(* Logix 5000 AddOnInstructionDefinition export Banner_EZAK2_Param_v4; software revision 33.00 *)

TYPE Banner_EZAK2_Channel_States_v4 :   // Channel States for the EZ-Array.
STRUCT
   State_16_to_1 : INT;
   State_32_to_17 : INT;
   State_48_to_33 : INT;
   State_64_to_49 : INT;
   State_80_to_65 : INT;
   State_96_to_81 : INT;
   State_112_to_97 : INT;
   State_128_to_113 : INT;
   State_144_to_129 : INT;
   State_160_to_145 : INT;
   State_176_to_161 : INT;
   State_192_to_177 : INT;
   State_208_to_193 : INT;
   State_224_to_209 : INT;
   State_240_to_225 : INT;
   State_256_to_241 : INT;
   State_272_to_257 : INT;
   State_288_to_273 : INT;
   State_304_to_289 : INT;
   State_320_to_305 : INT;
   State_336_to_321 : INT;
   State_352_to_337 : INT;
   State_368_to_353 : INT;
   State_384_to_369 : INT;
   State_400_to_385 : INT;
   State_416_to_401 : INT;
   State_432_to_417 : INT;
   State_448_to_433 : INT;
   State_464_to_449 : INT;
   State_480_to_465 : INT;
END_STRUCT
END_TYPE

TYPE Banner_EZAK2_RD_v4 :   // UDT with all of the Read only parameters for EZ-Array.
STRUCT
   Master_Cycle_Time : INT;
   Min_Cycle_Time : INT;
   M_Sequence_Capability : INT;
   IO_Link_Version_ID : INT;
   Process_Data_Input_Length : INT;
   Process_Data_Output_Length : INT;
   Combined_Vendor_ID : DINT;   // IO-Link Vendor ID
   Vendor_ID1 : INT;
   Vendor_ID2 : INT;
   Combined_Device_ID : DINT;   // IO-Link Device ID
   Device_ID1 : INT;
   Device_ID2 : INT;
   Device_ID3 : INT;
   Measurement_1 : DINT;
   Measurement_2 : DINT;
   CS : Banner_EZAK2_Channel_States_v4;   // Channel States
   Number_of_Emitter_Channels : DINT;
   Emitter_First_Bad_Channel : DINT;
   Number_of_Receiver_Channels : DINT;
   Dip_Switch_6 : SINT;   // 0 = ON, 1 = OFF
   Dip_Switch_5 : SINT;   // 0 = ON, 1 = OFF
   Dip_Switch_4 : SINT;   // 0 = ON, 1 = OFF
   Dip_Switch_3 : SINT;   // 0 = ON, 1 = OFF
   Dip_Switch_2 : SINT;   // 0 = ON, 1 = OFF
   Dip_Switch_1 : SINT;   // 0 = ON, 1 = OFF
   Error_Code : SINT;   // See IODD file for Error Codes.
   Alignment_Status : SINT;   // 0 = Failed, 1 = Success
   Discrete_Output_1 : SINT;   // 0 = OFF, 1 = ON
   Discrete_Output_2 : SINT;   // 0 = OFF, 1 = ON
   Analog_Output_1_DAC_Value : DINT;
   Analog_Output_2_DAC_Value : DINT;
   First_Beam_Blocked : DINT;
   Last_Beam_Blocked : DINT;
   Total_Beam_Blocked : DINT;
   Transitions : DINT;
   Contiguous_Beam_Blocked : DINT;
   First_Beam_Made : DINT;
   Last_Beam_Made : DINT;
   Total_Beam_Made : DINT;
   Contiguous_Beam_Made : DINT;
   Middle_Beam_Blocked : DINT;
   Outer_Diameter : DINT;
   Inner_Diameter : DINT;
   Contiguous_First_Beam_Blocked : DINT;
   Contiguous_Last_Beam_Blocked : DINT;
   Object_1_First_Beam_Blocked : DINT;
   Object_1_Last_Beam_Blocked : DINT;
   Object_2_First_Beam_Blocked : DINT;
   Object_2_Last_Beam_Blocked : DINT;
   Object_3_First_Beam_Blocked : DINT;
   Object_3_Last_Beam_Blocked : DINT;
   Carpet_Nap : DINT;
   Analog_1_Latched : DINT;
   Analog_2_Latched : DINT;
   Carpet_Edge : DINT;
   Receiver_Firmware_Number : DINT;
   Receiver_Firmware_Version : SINT;
   Emitter_Firmware_Number : DINT;
   Emitter_Firmware_Version : SINT;
   Communications_Fimware_Number : DINT;
   Communications_Firmware_Version : SINT;
END_STRUCT
END_TYPE

TYPE Banner_EZAK2_v4 :   // UDT with all of the parameters for EZ-Array.
STRUCT
   Initial_Global_Read : BOOL;   // Determines if all of the IO-Link data has been read into the PLC yet
   Command : INT;   // Value placed in here will activate a read or write to a specifc IO-Link Index
   Read : Banner_EZAK2_RD_v4;   // All read data
   Write : Banner_EZAK2_WD_v4;   // All data that can be written to.
   Archive_Data : Banner_EZAK2_WD_v4;
   Reset : BOOL;   // Resets AOI. This will force a complete parameter read of the sensor.
END_STRUCT
END_TYPE

TYPE Banner_EZAK2_WD_v4 :   // UDT that stores the Write Data for a EZ-Array.
STRUCT
   System_Command : INT;   // 130 = Factory Reset.
   Parameter_Access_Lock : SINT;
   Data_Storage_Lock : SINT;
   Local_Parameterization_Lock : SINT;
   Local_User_Interface_Lock : SINT;
   Scan_Type : INT;   // 1 = Straight, 2 = Single Edge, 3 = Double Edge (DE), 4 = DE Step 2, 5 = DE Step 4, 6 = DE Step 8, 7 = DE Step 16, 8=DE Step 32, 10 = Carpet Nap.
   Remote_Teach : INT;
   Blanking : Banner_EZAK2_Channel_States_v4;   // Status of Beam Banking
   Reserved : INT;
   Gain_Method : SINT;   // 1 = High Excess, 2 = Low Contrast
   Low_Contrast_Sensitivity : INT;
   Display_Orientation : SINT;   // 0 = Normal Orientation, 1 = Inverted Orientation
   Configuration_Type : SINT;   // 0 = Dip Switch Control, 1 = Advanced Control
   Sensitivity_Button : SINT;   // 0 = Enabled, 1 = Disabled
   Align_Blank_Button : SINT;   // 0 = Enabled, 1 = Disabled
   Measurement_1 : INT;   // 0=Disabled, 1=FBB, 2=LBB, 3=TBB, 4=TRN, 5=CBB, 6=FBM, 7=LBM, 8=TBM, 9=CBM, 10=MBB, 11=OD, 12=ID, 13=CFBB, 14=CLBB, 15=O1 FBB, 16=O1 LBB, 17=O2 FBB, 18=O2 LBB, 19=O3 FBB, 20=O3 LBB, 21=Carpet Nap, 24=Carpet Edge.
   Measurement_2 : INT;   // 0=Disabled, 1=FBB, 2=LBB, 3=TBB, 4=TRN, 5=CBB, 6=FBM, 7=LBM, 8=TBM, 9=CBM, 10=MBB, 11=OD, 12=ID, 13=CFBB, 14=CLBB, 15=O1 FBB, 16=O1 LBB, 17=O2 FBB, 18=O2 LBB, 19=O3 FBB, 20=O3 LBB, 21=Carpet Nap, 24=Carpet Edge.
   Number_of_Dirty_Channels : DINT;
   Time_of_Service : DINT;
   Alignment_Blanking_Mode : INT;   // 0=Status:Idle Mode, 1=Enter Align State, 2=Status:Align Mode, 3=Exit Align State, 4=Enter Blanking State, 5=Status: Blanking Mode, 6=Exit Blanking Mode.
   DO1_Status : SINT;   // 0 = Disabled, 1 = Enabled
   DO1_Type : SINT;   // 0 = Measurement Mode, 1 = Alarm or Health Mode
   DO1_Mode : SINT;   // 0 = NC (Alarm), 1 = NO (Health)
   DO1_Measurement : SINT;   // 0 = Measurement 2, 1 = Measurement 1
   DO1_Scan_Response : INT;   // See IODD for range.
   DO1_Hysteresis_Low : INT;   // See IODD for range.
   DO1_Hysteresis_High : INT;   // See IODD for range.
   DO1_Threshold_Low : INT;   // See IODD for range.
   DO1_Threshold_High : INT;   // See IODD for range.
   DO2_Status : SINT;   // 0 = Disabled, 1 = Enabled
   DO2_Type : SINT;   // 0 = Measurement Mode, 1 = Alarm or Health Mode
   DO2_Mode : SINT;   // 0 = NC (Alarm), 1 = NO (Health)
   DO2_Measurement : SINT;   // 0 = Measurement 2, 1 = Measurement 1
   DO2_Scan_Response : INT;   // See IODD for range.
   DO2_Hysteresis_Low : INT;   // See IODD for range.
   DO2_Hysteresis_High : INT;   // See IODD for range.
   DO2_Threshold_Low : INT;   // See IODD for range.
   DO2_Threshold_HIgh : INT;   // See IODD for range.
   Emitter_Power : INT;   // 1 to 11
   User_Process_Data : INT;   // 0 = Active Measurements, 1= Straight Scan, 2 = Single Double Edge, 128 = Channel States OR, 129 = Channel States AND.
   IO_Com : SINT;   // Allows for change between COM2 and Com3 Operation.
END_STRUCT
END_TYPE

TYPE Banner_IOL_Port_v4 :   // UDT that has all of the data items necessary to communicate with a specific Port on a IO-Link Master
STRUCT
   Port_Controlled : INT;   // Each bit represents a port on an IO-Link Master. Set to 1 to tell AOI to control that port.
   Port_Activate : INT;   // Each bit represents a port on an IO-Link Master. When ON that port will process any commands in queue.
   Port_Read : INT;   // Each bit represents a port on an IO-Link Master. Used to determine when device AOI has requested a Read command.
   Port_Write : INT;   // Each bit represents a port on an IO-Link Master. Used to determine when device AOI has requested a Write command.
   Port_RW_Complete : INT;   // Each bit represents a port on an IO-Link Master. Tells device AOI that Read or Write request has been completed.
   Port_Device_Read : INT;
   Data_Transfer : SINT[190];   // Array to transfer data from IO-Master to device AOIs.
END_STRUCT
END_TYPE

ADD_ON_INSTRUCTION Banner_EZAK2_Param_v4   (* revision 4.1, vendor Banner Engineering *)
// AOI to read and write parameter data to an IO-Link EZ-Array K2.
// Revision note:
// Fixed Alignment Blanking mode byte order for write. Switched System command from SINT to INT.
VAR_IN_OUT
   EZAK2 : Banner_EZAK2_v4; {required}
   Port_Data : Banner_IOL_Port_v4; {required}
END_VAR
VAR_INPUT
   Port : DINT; {required}
END_VAR
VAR
   Local_Control : DINT; {access None}
   Global_Read_Command_Value : INT; {access None}
   Global_Write_Command_Value : INT; {access None}
   Command_Being_Processed : BOOL; {access None}
   Update_Archive : BOOL; {access None}
   Index_Write_Control : DINT; {access None}
   Index_Write_Inprocess : INT; {access None}
   Inprocess_Index : DINT; {access None}
END_VAR

ROUTINE Logic   (* ladder *)
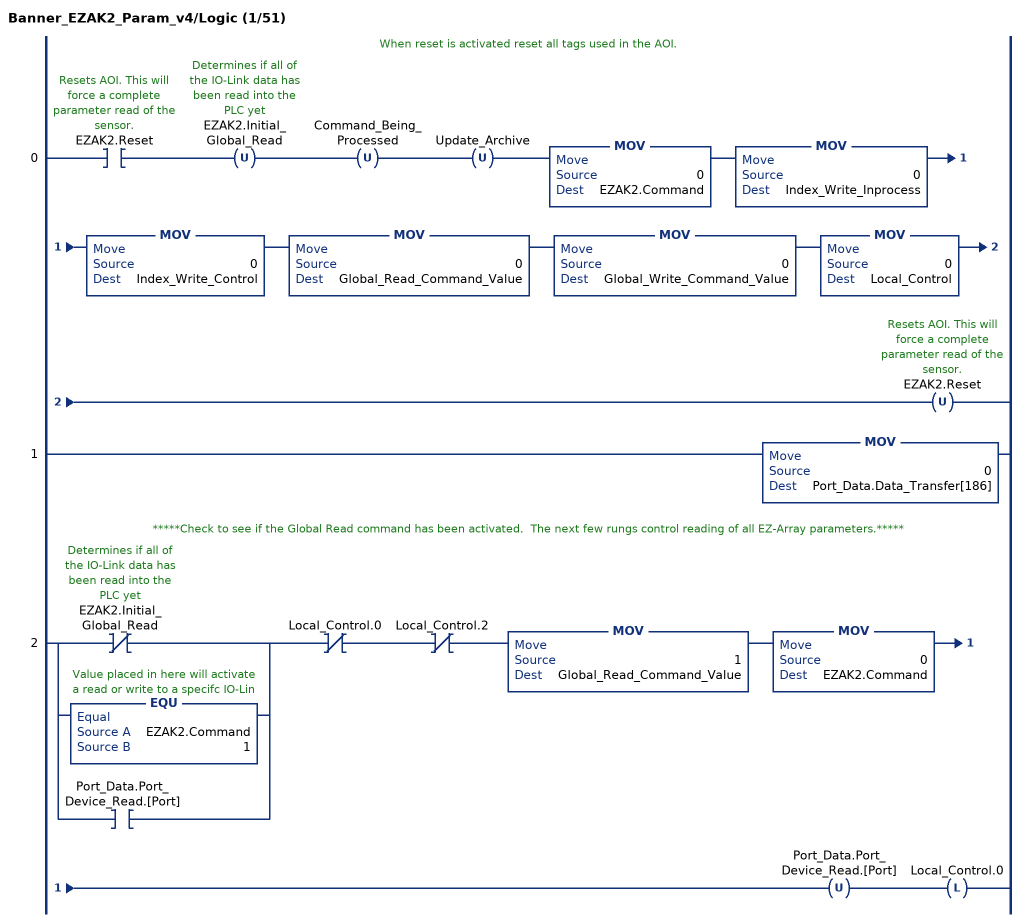
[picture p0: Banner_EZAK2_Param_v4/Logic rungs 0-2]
   // When reset is activated reset all tags used in the AOI.
   0: XIC(EZAK2.Reset)OTU(EZAK2.Initial_Global_Read)OTU(Command_Being_Processed)OTU(Update_Archive)MOV(0,EZAK2.Command)MOV(0,Index_Write_Inprocess)MOV(0,Index_Write_Control)MOV(0,Global_Read_Command_Value)MOV(0,Global_Write_Command_Value)MOV(0,Local_Control)OTU(EZAK2.Reset);
   1: MOV(0,Port_Data.Data_Transfer[186]);
   // *****Check to see if the Global Read command has been activated.  The next few rungs control reading of all EZ-Array parameters.*****
   2: [XIO(EZAK2.Initial_Global_Read) ,EQU(EZAK2.Command,1) ,XIC(Port_Data.Port_Device_Read.[Port]) ]XIO(Local_Control.0)XIO(Local_Control.2)MOV(1,Global_Read_Command_Value)MOV(0,EZAK2.Command)OTU(Port_Data.Port_Device_Read.[Port])OTL(Local_Control.0);
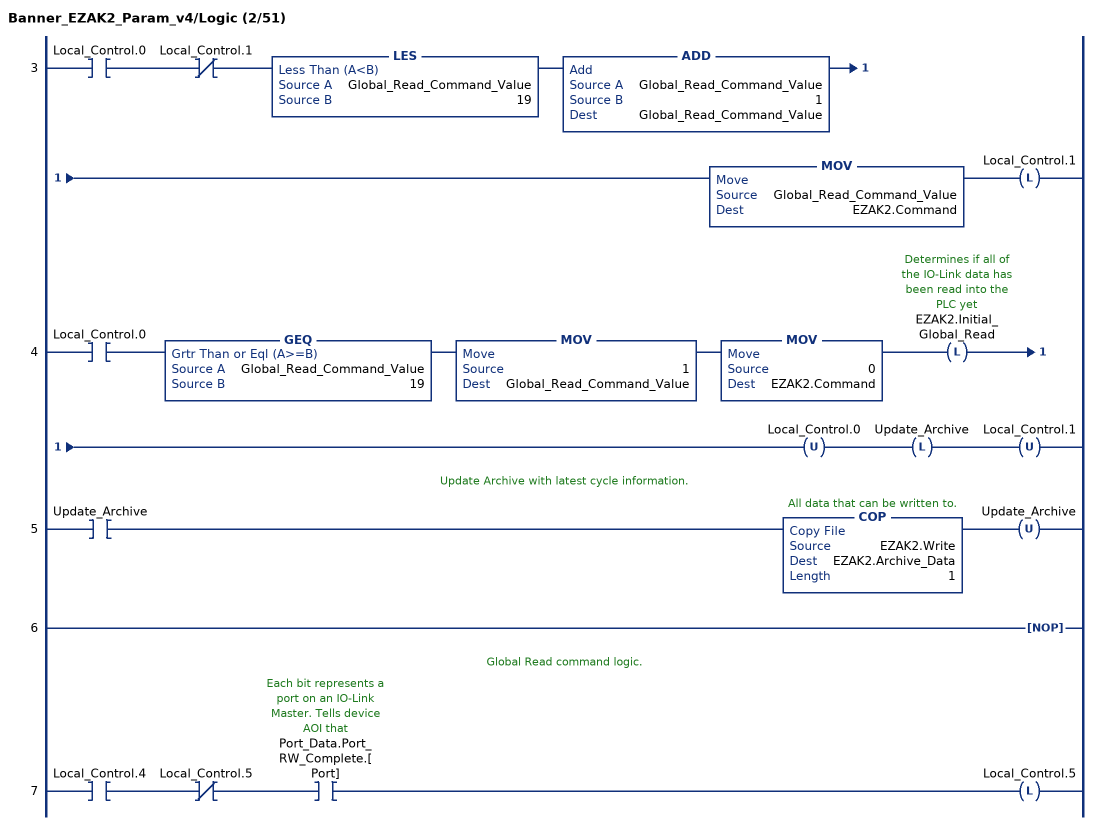
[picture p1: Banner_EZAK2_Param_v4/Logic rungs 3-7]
   3: XIC(Local_Control.0)XIO(Local_Control.1)LES(Global_Read_Command_Value,19)ADD(Global_Read_Command_Value,1,Global_Read_Command_Value)MOV(Global_Read_Command_Value,EZAK2.Command)OTL(Local_Control.1);
   4: XIC(Local_Control.0)GEQ(Global_Read_Command_Value,19)MOV(1,Global_Read_Command_Value)MOV(0,EZAK2.Command)OTL(EZAK2.Initial_Global_Read)OTU(Local_Control.0)OTL(Update_Archive)OTU(Local_Control.1);
   // Update Archive with latest cycle information.
   5: XIC(Update_Archive)COP(EZAK2.Write,EZAK2.Archive_Data,1)OTU(Update_Archive);
   6: NOP();
   // Global Read command logic.
   7: XIC(Local_Control.4)XIO(Local_Control.5)XIC(Port_Data.Port_RW_Complete.[Port])OTL(Local_Control.5);
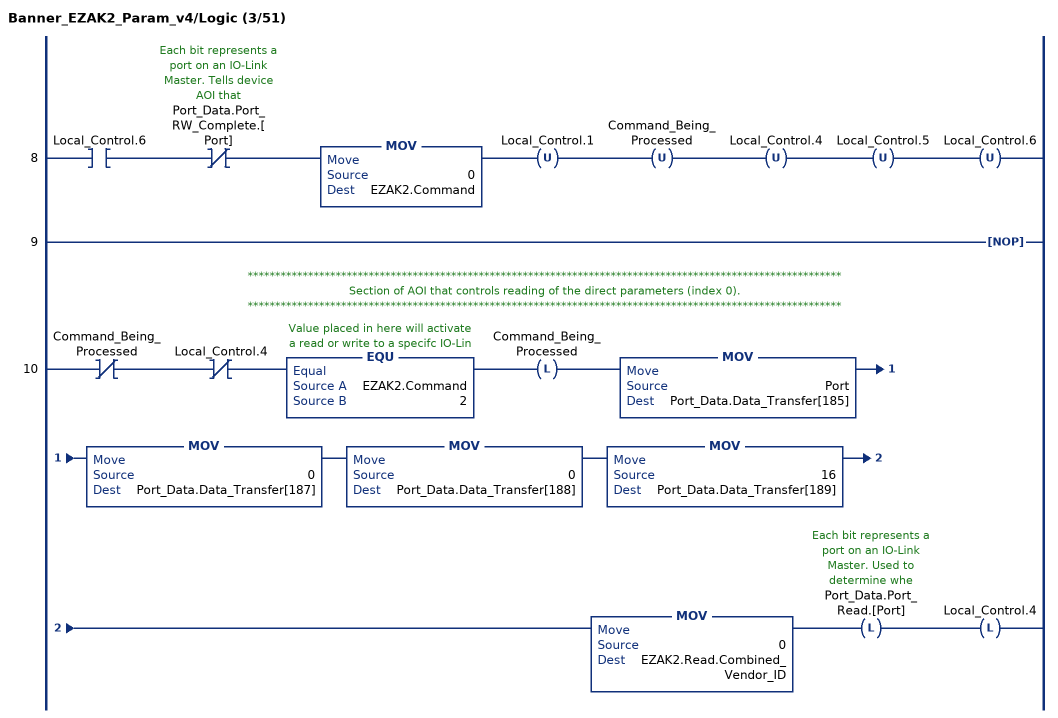
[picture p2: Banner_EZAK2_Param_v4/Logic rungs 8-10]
   8: XIC(Local_Control.6)XIO(Port_Data.Port_RW_Complete.[Port])MOV(0,EZAK2.Command)OTU(Local_Control.1)OTU(Command_Being_Processed)OTU(Local_Control.4)OTU(Local_Control.5)OTU(Local_Control.6);
   9: NOP();
   // ************************************************************************************************************
   // Section of AOI that controls reading of the direct parameters (index 0).
   // ************************************************************************************************************
   10: XIO(Command_Being_Processed)XIO(Local_Control.4)EQU(EZAK2.Command,2)OTL(Command_Being_Processed)MOV(Port,Port_Data.Data_Transfer[185])MOV(0,Port_Data.Data_Transfer[187])MOV(0,Port_Data.Data_Transfer[188])MOV(16,Port_Data.Data_Transfer[189])MOV(0,EZAK2.Read.Combined_Vendor_ID)OTL(Port_Data.Port_Read.[Port])OTL(Local_Control.4);
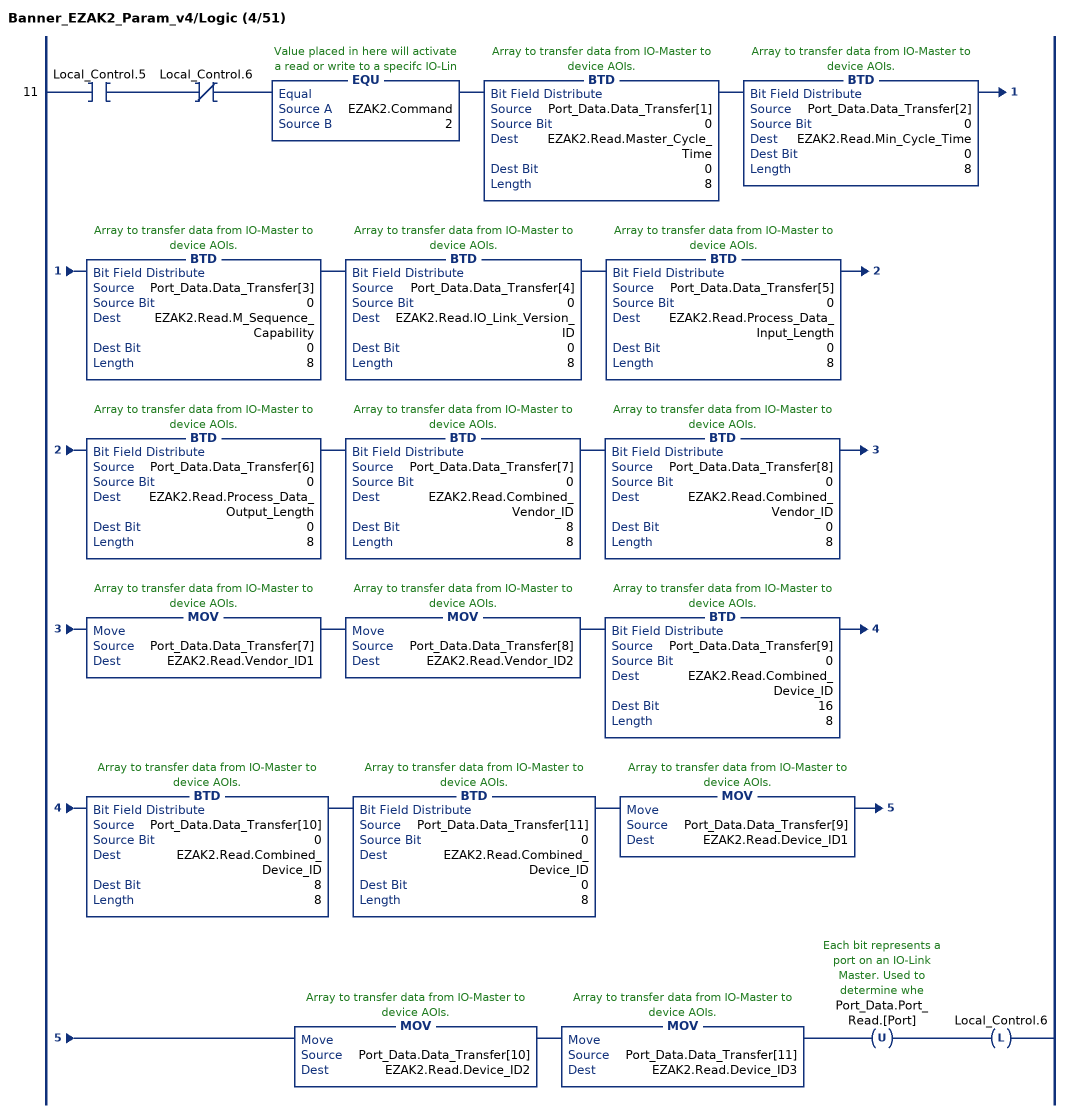
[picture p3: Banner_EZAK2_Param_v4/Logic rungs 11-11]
   11: XIC(Local_Control.5)XIO(Local_Control.6)EQU(EZAK2.Command,2)BTD(Port_Data.Data_Transfer[1],0,EZAK2.Read.Master_Cycle_Time,0,8)BTD(Port_Data.Data_Transfer[2],0,EZAK2.Read.Min_Cycle_Time,0,8)BTD(Port_Data.Data_Transfer[3],0,EZAK2.Read.M_Sequence_Capability,0,8)BTD(Port_Data.Data_Transfer[4],0,EZAK2.Read.IO_Link_Version_ID,0,8)BTD(Port_Data.Data_Transfer[5],0,EZAK2.Read.Process_Data_Input_Length,0,8)BTD(Port_Data.Data_Transfer[6],0,EZAK2.Read.Process_Data_Output_Length,0,8)BTD(Port_Data.Data_Transfer[7],0,EZAK2.Read.Combined_Vendor_ID,8,8)BTD(Port_Data.Data_Transfer[8],0,EZAK2.Read.Combined_Vendor_ID,0,8)MOV(Port_Data.Data_Transfer[7],EZAK2.Read.Vendor_ID1)MOV(Port_Data.Data_Transfer[8],EZAK2.Read.Vendor_ID2)BTD(Port_Data.Data_Transfer[9],0,EZAK2.Read.Combined_Device_ID,16,8)BTD(Port_Data.Data_Transfer[10],0,EZAK2.Read.Combined_Device_ID,8,8)BTD(Port_Data.Data_Transfer[11],0,EZAK2.Read.Combined_Device_ID,0,8)MOV(Port_Data.Data_Transfer[9],EZAK2.Read.Device_ID1)MOV(Port_Data.Data_Transfer[10],EZAK2.Read.Device_ID2)MOV(Port_Data.Data_Transfer[11],EZAK2.Read.Device_ID3)OTU(Port_Data.Port_Read.[Port])OTL(Local_Control.6);
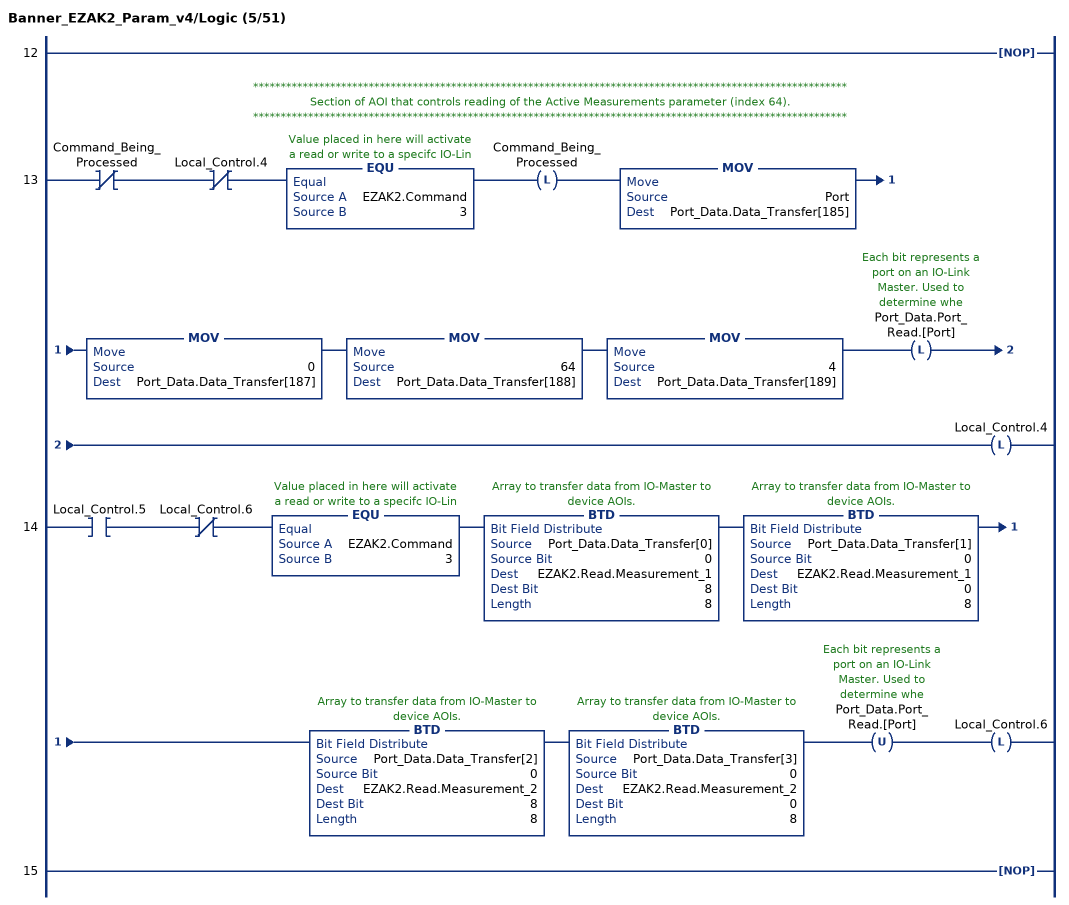
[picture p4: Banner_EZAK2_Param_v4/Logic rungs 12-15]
   12: NOP();
   // ************************************************************************************************************
   // Section of AOI that controls reading of the Active Measurements parameter (index 64).
   // ************************************************************************************************************
   13: XIO(Command_Being_Processed)XIO(Local_Control.4)EQU(EZAK2.Command,3)OTL(Command_Being_Processed)MOV(Port,Port_Data.Data_Transfer[185])MOV(0,Port_Data.Data_Transfer[187])MOV(64,Port_Data.Data_Transfer[188])MOV(4,Port_Data.Data_Transfer[189])OTL(Port_Data.Port_Read.[Port])OTL(Local_Control.4);
   14: XIC(Local_Control.5)XIO(Local_Control.6)EQU(EZAK2.Command,3)BTD(Port_Data.Data_Transfer[0],0,EZAK2.Read.Measurement_1,8,8)BTD(Port_Data.Data_Transfer[1],0,EZAK2.Read.Measurement_1,0,8)BTD(Port_Data.Data_Transfer[2],0,EZAK2.Read.Measurement_2,8,8)BTD(Port_Data.Data_Transfer[3],0,EZAK2.Read.Measurement_2,0,8)OTU(Port_Data.Port_Read.[Port])OTL(Local_Control.6);
   15: NOP();
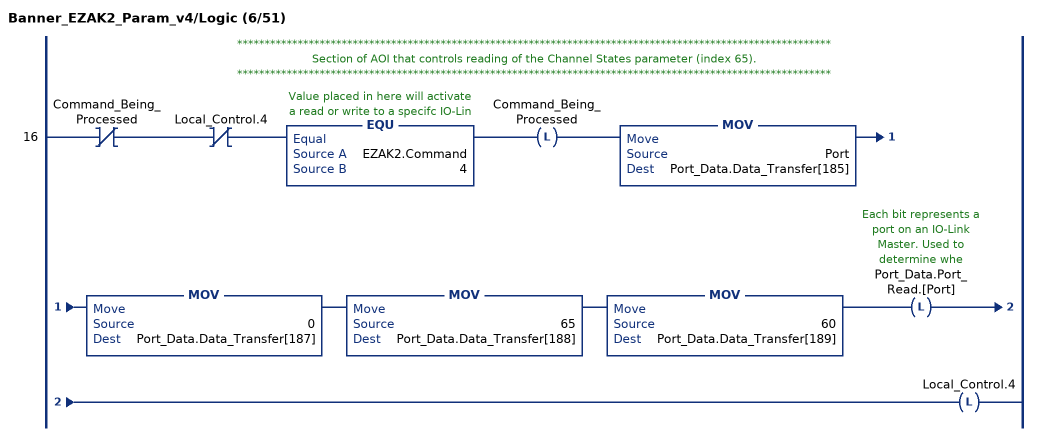
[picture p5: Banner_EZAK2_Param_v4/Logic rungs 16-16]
   // ************************************************************************************************************
   // Section of AOI that controls reading of the Channel States parameter (index 65).
   // ************************************************************************************************************
   16: XIO(Command_Being_Processed)XIO(Local_Control.4)EQU(EZAK2.Command,4)OTL(Command_Being_Processed)MOV(Port,Port_Data.Data_Transfer[185])MOV(0,Port_Data.Data_Transfer[187])MOV(65,Port_Data.Data_Transfer[188])MOV(60,Port_Data.Data_Transfer[189])OTL(Port_Data.Port_Read.[Port])OTL(Local_Control.4);
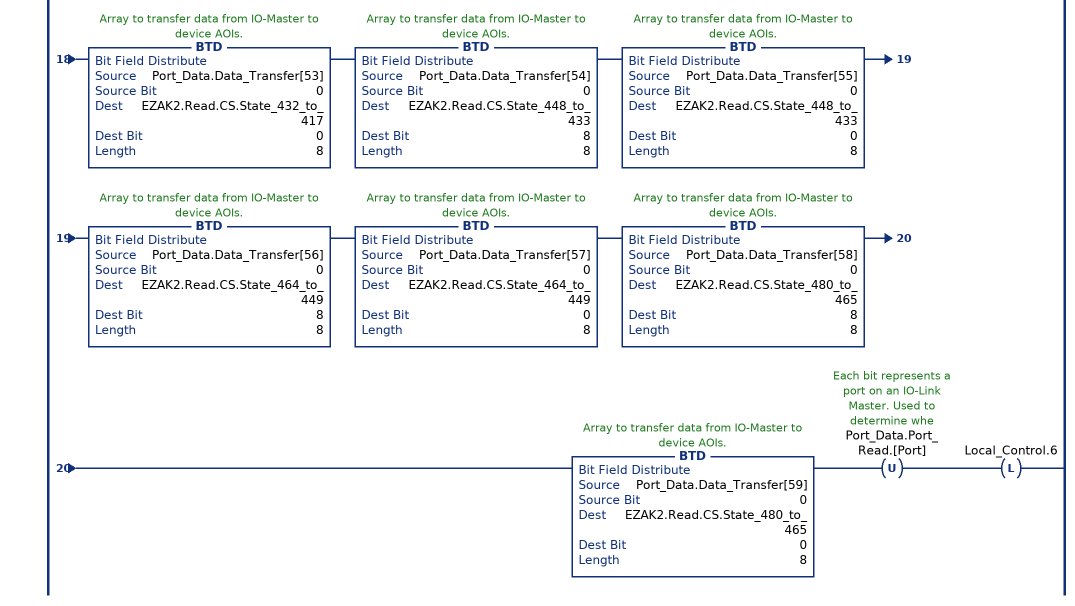
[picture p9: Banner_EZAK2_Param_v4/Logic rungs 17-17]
   17: XIC(Local_Control.5)XIO(Local_Control.6)EQU(EZAK2.Command,4)BTD(Port_Data.Data_Transfer[0],0,EZAK2.Read.CS.State_16_to_1,8,8)BTD(Port_Data.Data_Transfer[1],0,EZAK2.Read.CS.State_16_to_1,0,8)BTD(Port_Data.Data_Transfer[2],0,EZAK2.Read.CS.State_32_to_17,8,8)BTD(Port_Data.Data_Transfer[3],0,EZAK2.Read.CS.State_32_to_17,0,8)BTD(Port_Data.Data_Transfer[4],0,EZAK2.Read.CS.State_48_to_33,8,8)BTD(Port_Data.Data_Transfer[5],0,EZAK2.Read.CS.State_48_to_33,0,8)BTD(Port_Data.Data_Transfer[6],0,EZAK2.Read.CS.State_64_to_49,8,8)BTD(Port_Data.Data_Transfer[7],0,EZAK2.Read.CS.State_64_to_49,0,8)BTD(Port_Data.Data_Transfer[8],0,EZAK2.Read.CS.State_80_to_65,8,8)BTD(Port_Data.Data_Transfer[9],0,EZAK2.Read.CS.State_80_to_65,0,8)BTD(Port_Data.Data_Transfer[10],0,EZAK2.Read.CS.State_96_to_81,8,8)BTD(Port_Data.Data_Transfer[11],0,EZAK2.Read.CS.State_96_to_81,0,8)BTD(Port_Data.Data_Transfer[12],0,EZAK2.Read.CS.State_112_to_97,8,8)BTD(Port_Data.Data_Transfer[13],0,EZAK2.Read.CS.State_112_to_97,0,8)BTD(Port_Data.Data_Transfer[14],0,EZAK2.Read.CS.State_128_to_113,8,8)BTD(Port_Data.Data_Transfer[15],0,EZAK2.Read.CS.State_128_to_113,0,8)BTD(Port_Data.Data_Transfer[16],0,EZAK2.Read.CS.State_144_to_129,8,8)BTD(Port_Data.Data_Transfer[17],0,EZAK2.Read.CS.State_144_to_129,0,8)BTD(Port_Data.Data_Transfer[18],0,EZAK2.Read.CS.State_160_to_145,8,8)BTD(Port_Data.Data_Transfer[19],0,EZAK2.Read.CS.State_160_to_145,0,8)BTD(Port_Data.Data_Transfer[20],0,EZAK2.Read.CS.State_176_to_161,8,8)BTD(Port_Data.Data_Transfer[21],0,EZAK2.Read.CS.State_176_to_161,0,8)BTD(Port_Data.Data_Transfer[22],0,EZAK2.Read.CS.State_192_to_177,8,8)BTD(Port_Data.Data_Transfer[23],0,EZAK2.Read.CS.State_192_to_177,0,8)BTD(Port_Data.Data_Transfer[24],0,EZAK2.Read.CS.State_208_to_193,8,8)BTD(Port_Data.Data_Transfer[25],0,EZAK2.Read.CS.State_208_to_193,0,8)BTD(Port_Data.Data_Transfer[26],0,EZAK2.Read.CS.State_224_to_209,8,8)BTD(Port_Data.Data_Transfer[27],0,EZAK2.Read.CS.State_224_to_209,0,8)BTD(Port_Data.Data_Transfer[28],0,EZAK2.Read.CS.State_240_to_225,8,8)BTD(Port_Data.Data_Transfer[29],0,EZAK2.Read.CS.State_240_to_225,0,8)BTD(Port_Data.Data_Transfer[30],0,EZAK2.Read.CS.State_256_to_241,8,8)BTD(Port_Data.Data_Transfer[31],0,EZAK2.Read.CS.State_256_to_241,0,8)BTD(Port_Data.Data_Transfer[32],0,EZAK2.Read.CS.State_272_to_257,8,8)BTD(Port_Data.Data_Transfer[33],0,EZAK2.Read.CS.State_272_to_257,0,8)BTD(Port_Data.Data_Transfer[34],0,EZAK2.Read.CS.State_288_to_273,8,8)BTD(Port_Data.Data_Transfer[35],0,EZAK2.Read.CS.State_288_to_273,0,8)BTD(Port_Data.Data_Transfer[36],0,EZAK2.Read.CS.State_304_to_289,8,8)BTD(Port_Data.Data_Transfer[37],0,EZAK2.Read.CS.State_304_to_289,0,8)BTD(Port_Data.Data_Transfer[38],0,EZAK2.Read.CS.State_320_to_305,8,8)BTD(Port_Data.Data_Transfer[39],0,EZAK2.Read.CS.State_320_to_305,0,8)BTD(Port_Data.Data_Transfer[40],0,EZAK2.Read.CS.State_336_to_321,8,8)BTD(Port_Data.Data_Transfer[41],0,EZAK2.Read.CS.State_336_to_321,0,8)BTD(Port_Data.Data_Transfer[42],0,EZAK2.Read.CS.State_352_to_337,8,8)BTD(Port_Data.Data_Transfer[43],0,EZAK2.Read.CS.State_352_to_337,0,8)BTD(Port_Data.Data_Transfer[44],0,EZAK2.Read.CS.State_368_to_353,8,8)BTD(Port_Data.Data_Transfer[45],0,EZAK2.Read.CS.State_368_to_353,0,8)BTD(Port_Data.Data_Transfer[46],0,EZAK2.Read.CS.State_384_to_369,8,8)BTD(Port_Data.Data_Transfer[47],0,EZAK2.Read.CS.State_384_to_369,0,8)BTD(Port_Data.Data_Transfer[48],0,EZAK2.Read.CS.State_400_to_385,8,8)BTD(Port_Data.Data_Transfer[49],0,EZAK2.Read.CS.State_400_to_385,0,8)BTD(Port_Data.Data_Transfer[50],0,EZAK2.Read.CS.State_416_to_401,8,8)BTD(Port_Data.Data_Transfer[51],0,EZAK2.Read.CS.State_416_to_401,0,8)BTD(Port_Data.Data_Transfer[52],0,EZAK2.Read.CS.State_432_to_417,8,8)BTD(Port_Data.Data_Transfer[53],0,EZAK2.Read.CS.State_432_to_417,0,8)BTD(Port_Data.Data_Transfer[54],0,EZAK2.Read.CS.State_448_to_433,8,8)BTD(Port_Data.Data_Transfer[55],0,EZAK2.Read.CS.State_448_to_433,0,8)BTD(Port_Data.Data_Transfer[56],0,EZAK2.Read.CS.State_464_to_449,8,8)BTD(Port_Data.Data_Transfer[57],0,EZAK2.Read.CS.State_464_to_449,0,8)BTD(Port_Data.Data_Transfer[58],0,EZAK2.Read.CS.State_480_to_465,8,8)BTD(Port_Data.Data_Transfer[59],0,EZAK2.Read.CS.State_480_to_465,0,8)OTU(Port_Data.Port_Read.[Port])OTL(Local_Control.6);
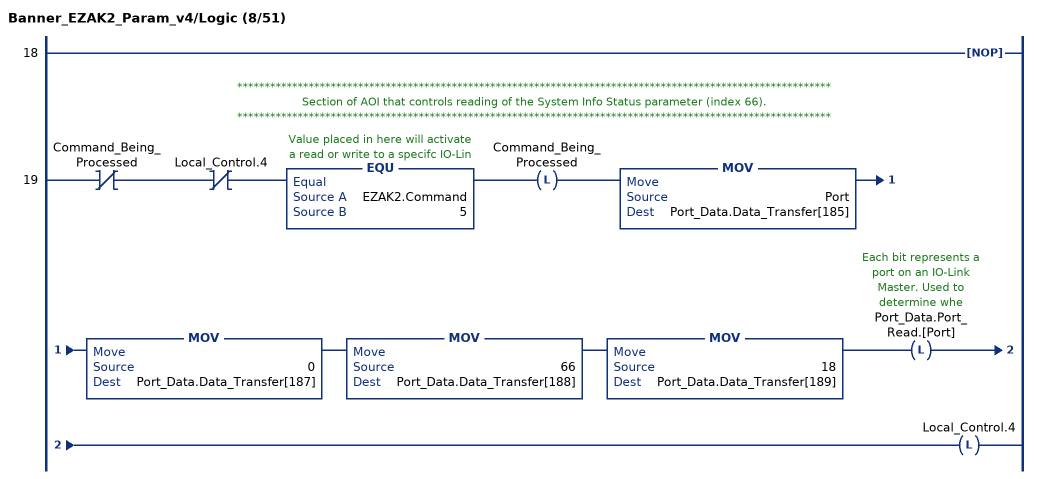
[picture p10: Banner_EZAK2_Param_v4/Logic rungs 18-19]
   18: NOP();
   // ************************************************************************************************************
   // Section of AOI that controls reading of the System Info Status parameter (index 66).
   // ************************************************************************************************************
   19: XIO(Command_Being_Processed)XIO(Local_Control.4)EQU(EZAK2.Command,5)OTL(Command_Being_Processed)MOV(Port,Port_Data.Data_Transfer[185])MOV(0,Port_Data.Data_Transfer[187])MOV(66,Port_Data.Data_Transfer[188])MOV(18,Port_Data.Data_Transfer[189])OTL(Port_Data.Port_Read.[Port])OTL(Local_Control.4);
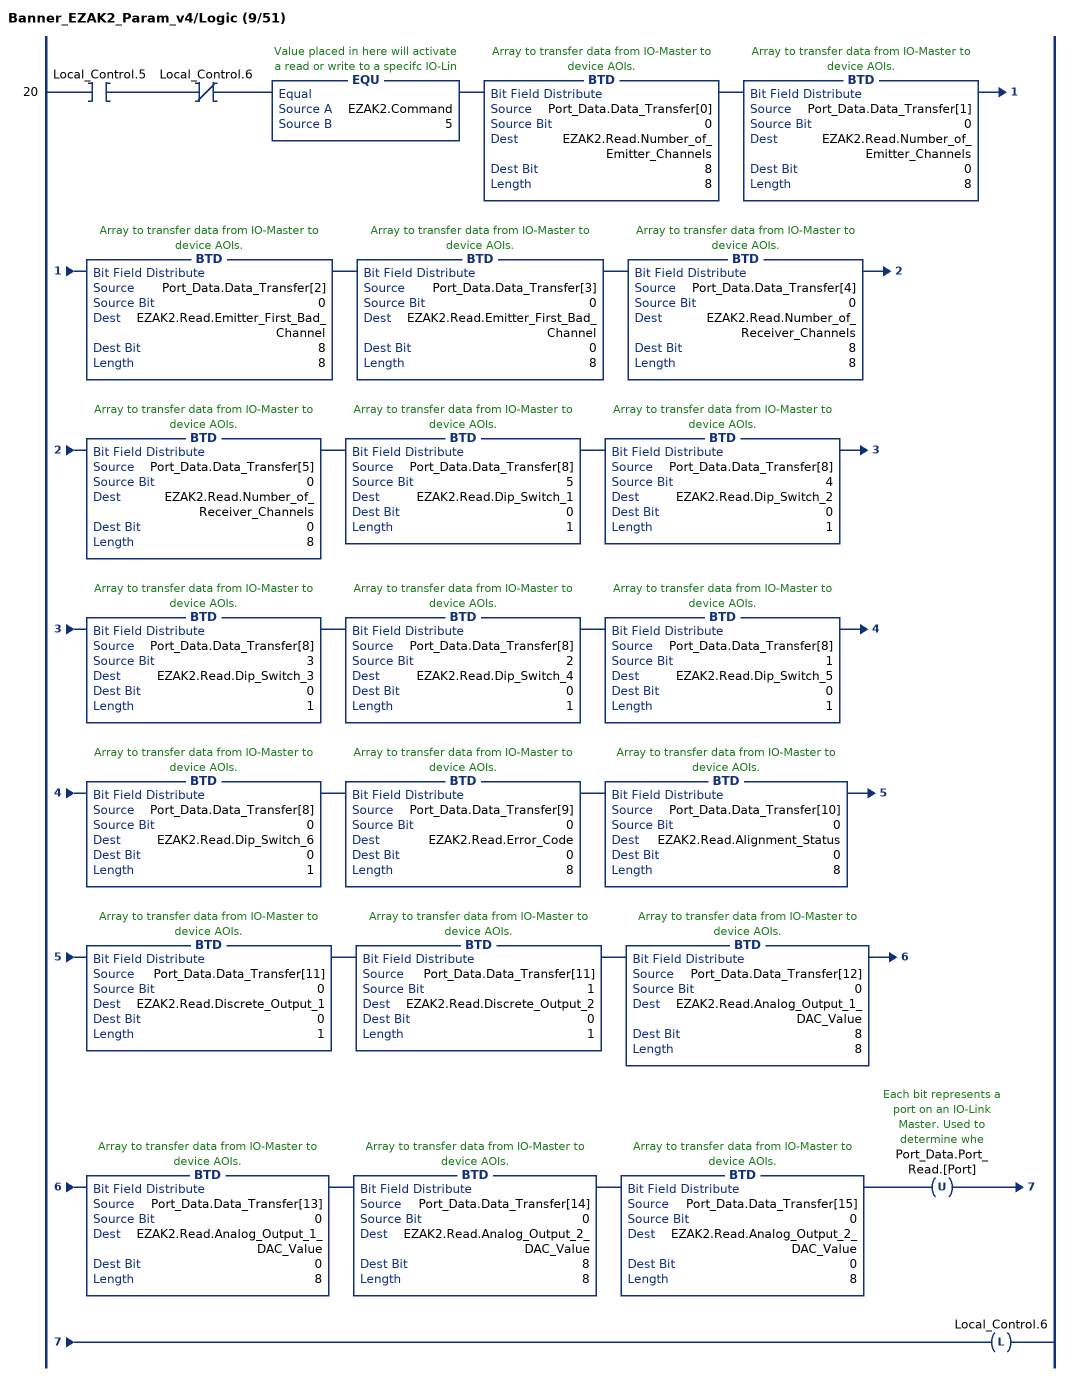
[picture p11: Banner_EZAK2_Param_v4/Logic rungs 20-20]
   20: XIC(Local_Control.5)XIO(Local_Control.6)EQU(EZAK2.Command,5)BTD(Port_Data.Data_Transfer[0],0,EZAK2.Read.Number_of_Emitter_Channels,8,8)BTD(Port_Data.Data_Transfer[1],0,EZAK2.Read.Number_of_Emitter_Channels,0,8)BTD(Port_Data.Data_Transfer[2],0,EZAK2.Read.Emitter_First_Bad_Channel,8,8)BTD(Port_Data.Data_Transfer[3],0,EZAK2.Read.Emitter_First_Bad_Channel,0,8)BTD(Port_Data.Data_Transfer[4],0,EZAK2.Read.Number_of_Receiver_Channels,8,8)BTD(Port_Data.Data_Transfer[5],0,EZAK2.Read.Number_of_Receiver_Channels,0,8)BTD(Port_Data.Data_Transfer[8],5,EZAK2.Read.Dip_Switch_1,0,1)BTD(Port_Data.Data_Transfer[8],4,EZAK2.Read.Dip_Switch_2,0,1)BTD(Port_Data.Data_Transfer[8],3,EZAK2.Read.Dip_Switch_3,0,1)BTD(Port_Data.Data_Transfer[8],2,EZAK2.Read.Dip_Switch_4,0,1)BTD(Port_Data.Data_Transfer[8],1,EZAK2.Read.Dip_Switch_5,0,1)BTD(Port_Data.Data_Transfer[8],0,EZAK2.Read.Dip_Switch_6,0,1)BTD(Port_Data.Data_Transfer[9],0,EZAK2.Read.Error_Code,0,8)BTD(Port_Data.Data_Transfer[10],0,EZAK2.Read.Alignment_Status,0,8)BTD(Port_Data.Data_Transfer[11],0,EZAK2.Read.Discrete_Output_1,0,1)BTD(Port_Data.Data_Transfer[11],1,EZAK2.Read.Discrete_Output_2,0,1)BTD(Port_Data.Data_Transfer[12],0,EZAK2.Read.Analog_Output_1_DAC_Value,8,8)BTD(Port_Data.Data_Transfer[13],0,EZAK2.Read.Analog_Output_1_DAC_Value,0,8)BTD(Port_Data.Data_Transfer[14],0,EZAK2.Read.Analog_Output_2_DAC_Value,8,8)BTD(Port_Data.Data_Transfer[15],0,EZAK2.Read.Analog_Output_2_DAC_Value,0,8)OTU(Port_Data.Port_Read.[Port])OTL(Local_Control.6);
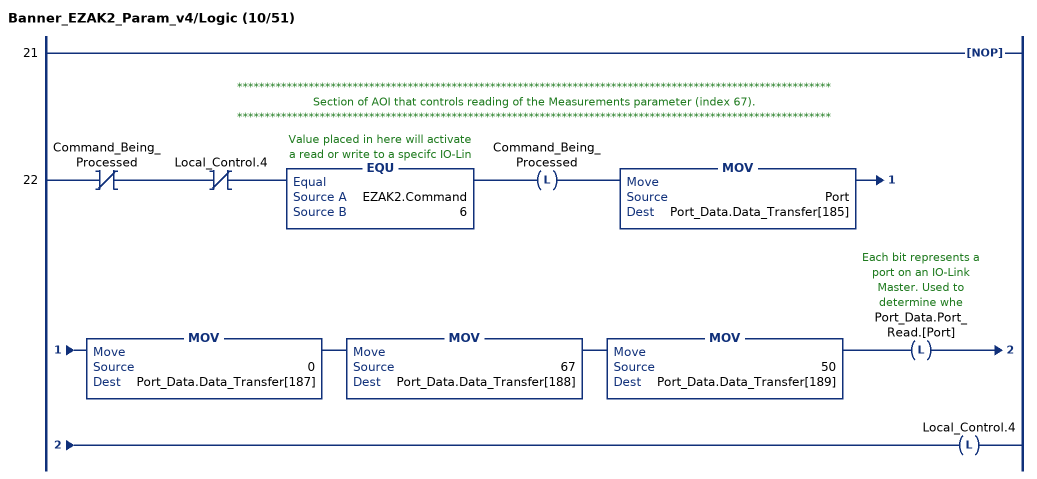
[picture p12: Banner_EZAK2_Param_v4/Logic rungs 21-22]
   21: NOP();
   // ************************************************************************************************************
   // Section of AOI that controls reading of the Measurements parameter (index 67).
   // ************************************************************************************************************
   22: XIO(Command_Being_Processed)XIO(Local_Control.4)EQU(EZAK2.Command,6)OTL(Command_Being_Processed)MOV(Port,Port_Data.Data_Transfer[185])MOV(0,Port_Data.Data_Transfer[187])MOV(67,Port_Data.Data_Transfer[188])MOV(50,Port_Data.Data_Transfer[189])OTL(Port_Data.Port_Read.[Port])OTL(Local_Control.4);
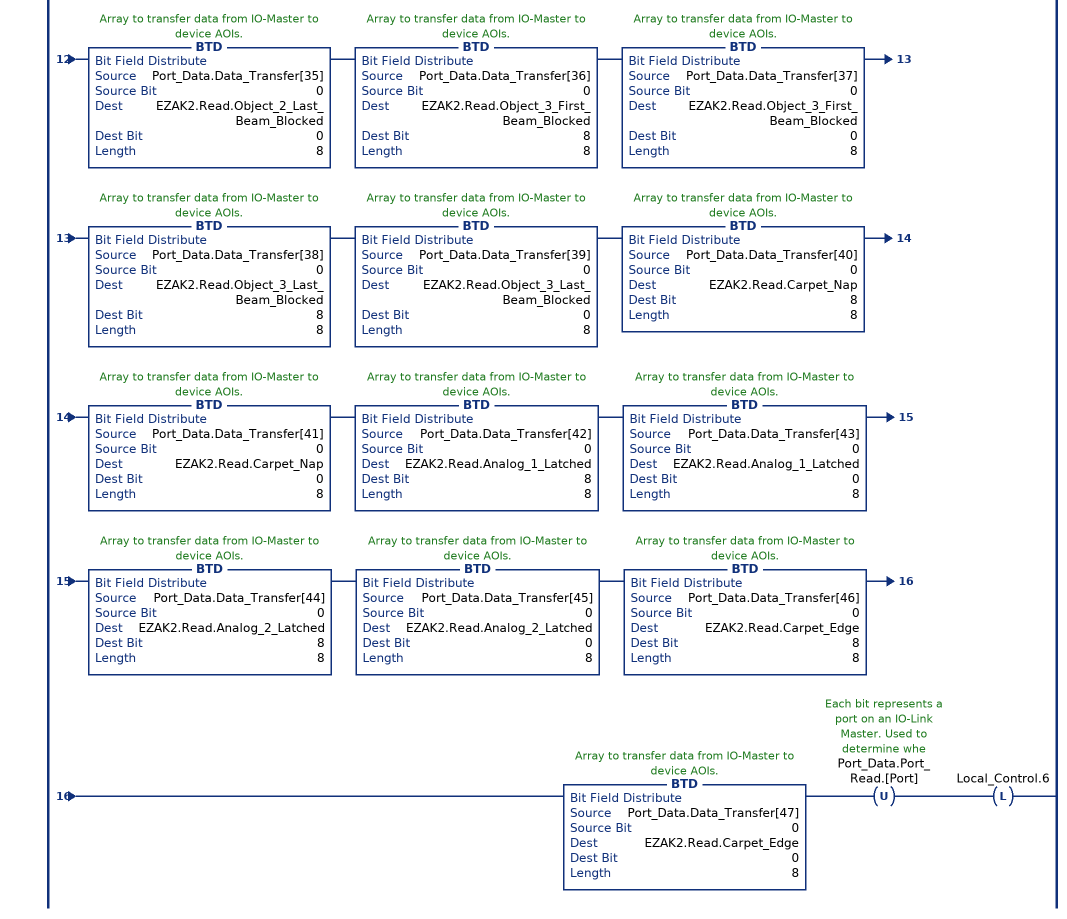
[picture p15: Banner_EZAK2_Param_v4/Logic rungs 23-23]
   23: XIC(Local_Control.5)XIO(Local_Control.6)EQU(EZAK2.Command,6)BTD(Port_Data.Data_Transfer[0],0,EZAK2.Read.First_Beam_Blocked,8,8)BTD(Port_Data.Data_Transfer[1],0,EZAK2.Read.First_Beam_Blocked,0,8)BTD(Port_Data.Data_Transfer[2],0,EZAK2.Read.Last_Beam_Blocked,8,8)BTD(Port_Data.Data_Transfer[3],0,EZAK2.Read.Last_Beam_Blocked,0,8)BTD(Port_Data.Data_Transfer[4],0,EZAK2.Read.Total_Beam_Blocked,8,8)BTD(Port_Data.Data_Transfer[5],0,EZAK2.Read.Total_Beam_Blocked,0,8)BTD(Port_Data.Data_Transfer[6],0,EZAK2.Read.Transitions,8,8)BTD(Port_Data.Data_Transfer[7],0,EZAK2.Read.Transitions,0,8)BTD(Port_Data.Data_Transfer[8],0,EZAK2.Read.Contiguous_Beam_Blocked,8,8)BTD(Port_Data.Data_Transfer[9],0,EZAK2.Read.Contiguous_Beam_Blocked,0,8)BTD(Port_Data.Data_Transfer[10],0,EZAK2.Read.First_Beam_Made,8,8)BTD(Port_Data.Data_Transfer[11],0,EZAK2.Read.First_Beam_Made,0,8)BTD(Port_Data.Data_Transfer[12],0,EZAK2.Read.Last_Beam_Made,8,8)BTD(Port_Data.Data_Transfer[13],0,EZAK2.Read.Last_Beam_Made,0,8)BTD(Port_Data.Data_Transfer[14],0,EZAK2.Read.Total_Beam_Made,8,8)BTD(Port_Data.Data_Transfer[15],0,EZAK2.Read.Total_Beam_Made,0,8)BTD(Port_Data.Data_Transfer[16],0,EZAK2.Read.Contiguous_Beam_Made,8,8)BTD(Port_Data.Data_Transfer[17],0,EZAK2.Read.Contiguous_Beam_Made,0,8)BTD(Port_Data.Data_Transfer[18],0,EZAK2.Read.Middle_Beam_Blocked,8,8)BTD(Port_Data.Data_Transfer[19],0,EZAK2.Read.Middle_Beam_Blocked,0,8)BTD(Port_Data.Data_Transfer[20],0,EZAK2.Read.Outer_Diameter,8,8)BTD(Port_Data.Data_Transfer[21],0,EZAK2.Read.Outer_Diameter,0,8)BTD(Port_Data.Data_Transfer[22],0,EZAK2.Read.Inner_Diameter,8,8)BTD(Port_Data.Data_Transfer[23],0,EZAK2.Read.Inner_Diameter,0,8)BTD(Port_Data.Data_Transfer[24],0,EZAK2.Read.Contiguous_First_Beam_Blocked,8,8)BTD(Port_Data.Data_Transfer[25],0,EZAK2.Read.Contiguous_First_Beam_Blocked,0,8)BTD(Port_Data.Data_Transfer[26],0,EZAK2.Read.Contiguous_Last_Beam_Blocked,8,8)BTD(Port_Data.Data_Transfer[27],0,EZAK2.Read.Contiguous_Last_Beam_Blocked,0,8)BTD(Port_Data.Data_Transfer[28],0,EZAK2.Read.Object_1_First_Beam_Blocked,8,8)BTD(Port_Data.Data_Transfer[29],0,EZAK2.Read.Object_1_First_Beam_Blocked,0,8)BTD(Port_Data.Data_Transfer[30],0,EZAK2.Read.Object_1_Last_Beam_Blocked,8,8)BTD(Port_Data.Data_Transfer[31],0,EZAK2.Read.Object_1_Last_Beam_Blocked,0,8)BTD(Port_Data.Data_Transfer[32],0,EZAK2.Read.Object_2_First_Beam_Blocked,8,8)BTD(Port_Data.Data_Transfer[33],0,EZAK2.Read.Object_2_First_Beam_Blocked,0,8)BTD(Port_Data.Data_Transfer[34],0,EZAK2.Read.Object_2_Last_Beam_Blocked,8,8)BTD(Port_Data.Data_Transfer[35],0,EZAK2.Read.Object_2_Last_Beam_Blocked,0,8)BTD(Port_Data.Data_Transfer[36],0,EZAK2.Read.Object_3_First_Beam_Blocked,8,8)BTD(Port_Data.Data_Transfer[37],0,EZAK2.Read.Object_3_First_Beam_Blocked,0,8)BTD(Port_Data.Data_Transfer[38],0,EZAK2.Read.Object_3_Last_Beam_Blocked,8,8)BTD(Port_Data.Data_Transfer[39],0,EZAK2.Read.Object_3_Last_Beam_Blocked,0,8)BTD(Port_Data.Data_Transfer[40],0,EZAK2.Read.Carpet_Nap,8,8)BTD(Port_Data.Data_Transfer[41],0,EZAK2.Read.Carpet_Nap,0,8)BTD(Port_Data.Data_Transfer[42],0,EZAK2.Read.Analog_1_Latched,8,8)BTD(Port_Data.Data_Transfer[43],0,EZAK2.Read.Analog_1_Latched,0,8)BTD(Port_Data.Data_Transfer[44],0,EZAK2.Read.Analog_2_Latched,8,8)BTD(Port_Data.Data_Transfer[45],0,EZAK2.Read.Analog_2_Latched,0,8)BTD(Port_Data.Data_Transfer[46],0,EZAK2.Read.Carpet_Edge,8,8)BTD(Port_Data.Data_Transfer[47],0,EZAK2.Read.Carpet_Edge,0,8)OTU(Port_Data.Port_Read.[Port])OTL(Local_Control.6);
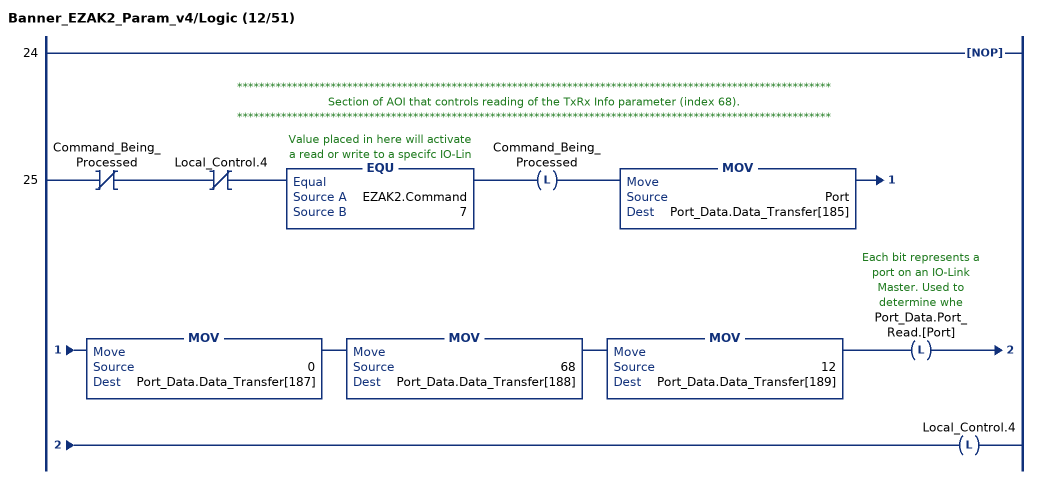
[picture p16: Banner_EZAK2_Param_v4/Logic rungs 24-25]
   24: NOP();
   // ************************************************************************************************************
   // Section of AOI that controls reading of the TxRx Info parameter (index 68).
   // ************************************************************************************************************
   25: XIO(Command_Being_Processed)XIO(Local_Control.4)EQU(EZAK2.Command,7)OTL(Command_Being_Processed)MOV(Port,Port_Data.Data_Transfer[185])MOV(0,Port_Data.Data_Transfer[187])MOV(68,Port_Data.Data_Transfer[188])MOV(12,Port_Data.Data_Transfer[189])OTL(Port_Data.Port_Read.[Port])OTL(Local_Control.4);
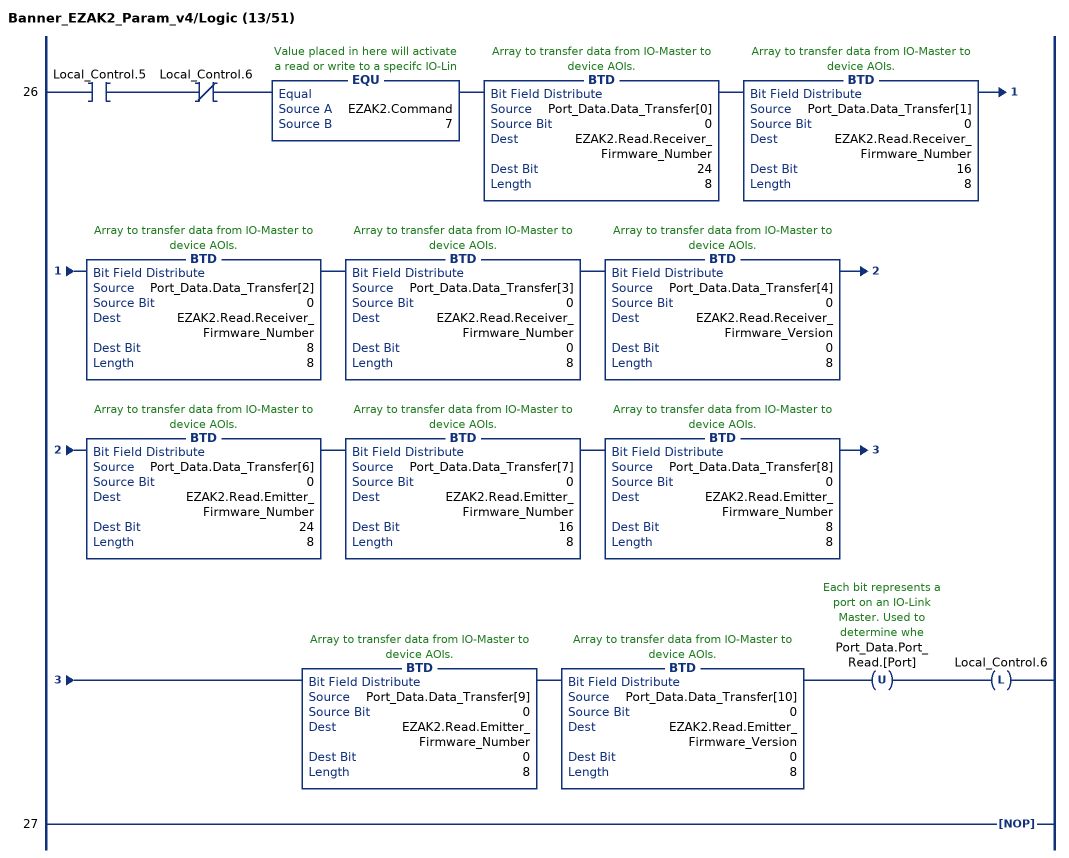
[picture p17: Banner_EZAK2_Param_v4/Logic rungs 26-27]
   26: XIC(Local_Control.5)XIO(Local_Control.6)EQU(EZAK2.Command,7)BTD(Port_Data.Data_Transfer[0],0,EZAK2.Read.Receiver_Firmware_Number,24,8)BTD(Port_Data.Data_Transfer[1],0,EZAK2.Read.Receiver_Firmware_Number,16,8)BTD(Port_Data.Data_Transfer[2],0,EZAK2.Read.Receiver_Firmware_Number,8,8)BTD(Port_Data.Data_Transfer[3],0,EZAK2.Read.Receiver_Firmware_Number,0,8)BTD(Port_Data.Data_Transfer[4],0,EZAK2.Read.Receiver_Firmware_Version,0,8)BTD(Port_Data.Data_Transfer[6],0,EZAK2.Read.Emitter_Firmware_Number,24,8)BTD(Port_Data.Data_Transfer[7],0,EZAK2.Read.Emitter_Firmware_Number,16,8)BTD(Port_Data.Data_Transfer[8],0,EZAK2.Read.Emitter_Firmware_Number,8,8)BTD(Port_Data.Data_Transfer[9],0,EZAK2.Read.Emitter_Firmware_Number,0,8)BTD(Port_Data.Data_Transfer[10],0,EZAK2.Read.Emitter_Firmware_Version,0,8)OTU(Port_Data.Port_Read.[Port])OTL(Local_Control.6);
   27: NOP();
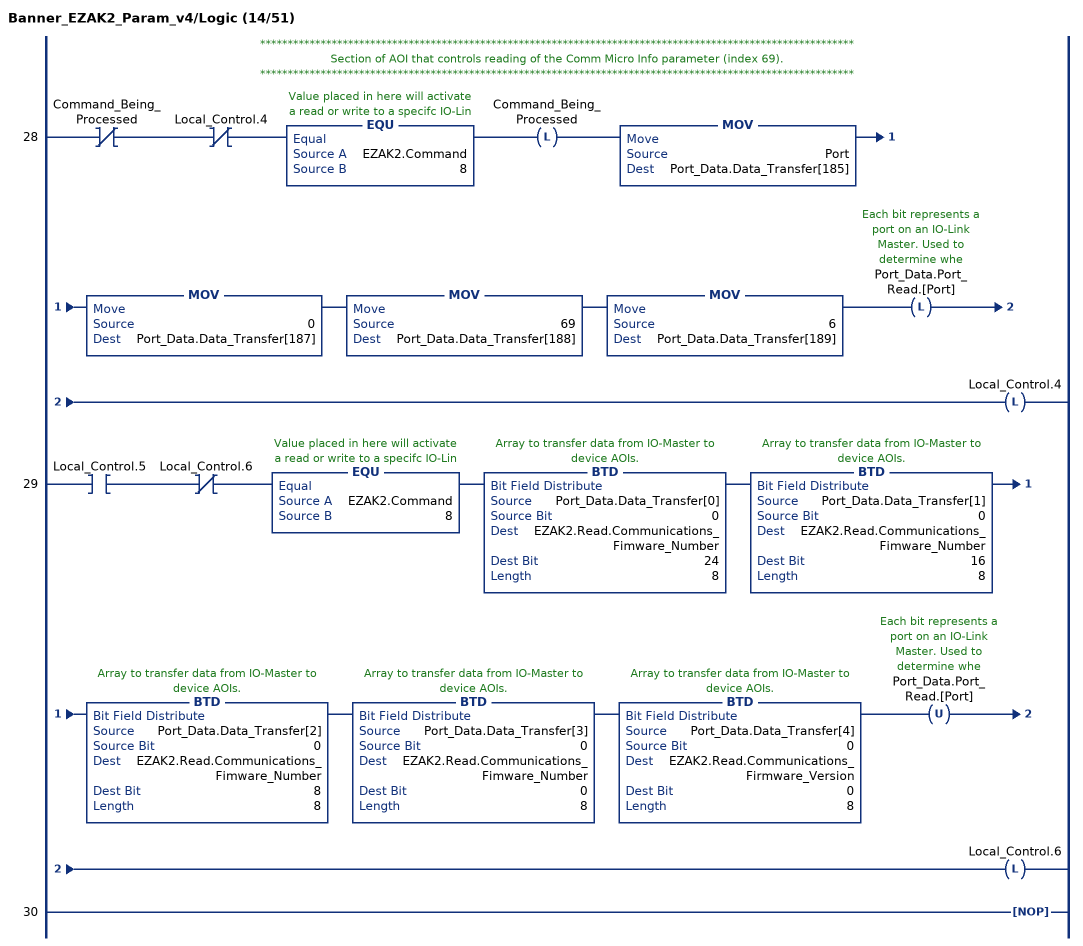
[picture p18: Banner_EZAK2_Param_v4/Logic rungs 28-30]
   // ************************************************************************************************************
   // Section of AOI that controls reading of the Comm Micro Info parameter (index 69).
   // ************************************************************************************************************
   28: XIO(Command_Being_Processed)XIO(Local_Control.4)EQU(EZAK2.Command,8)OTL(Command_Being_Processed)MOV(Port,Port_Data.Data_Transfer[185])MOV(0,Port_Data.Data_Transfer[187])MOV(69,Port_Data.Data_Transfer[188])MOV(6,Port_Data.Data_Transfer[189])OTL(Port_Data.Port_Read.[Port])OTL(Local_Control.4);
   29: XIC(Local_Control.5)XIO(Local_Control.6)EQU(EZAK2.Command,8)BTD(Port_Data.Data_Transfer[0],0,EZAK2.Read.Communications_Fimware_Number,24,8)BTD(Port_Data.Data_Transfer[1],0,EZAK2.Read.Communications_Fimware_Number,16,8)BTD(Port_Data.Data_Transfer[2],0,EZAK2.Read.Communications_Fimware_Number,8,8)BTD(Port_Data.Data_Transfer[3],0,EZAK2.Read.Communications_Fimware_Number,0,8)BTD(Port_Data.Data_Transfer[4],0,EZAK2.Read.Communications_Firmware_Version,0,8)OTU(Port_Data.Port_Read.[Port])OTL(Local_Control.6);
   30: NOP();
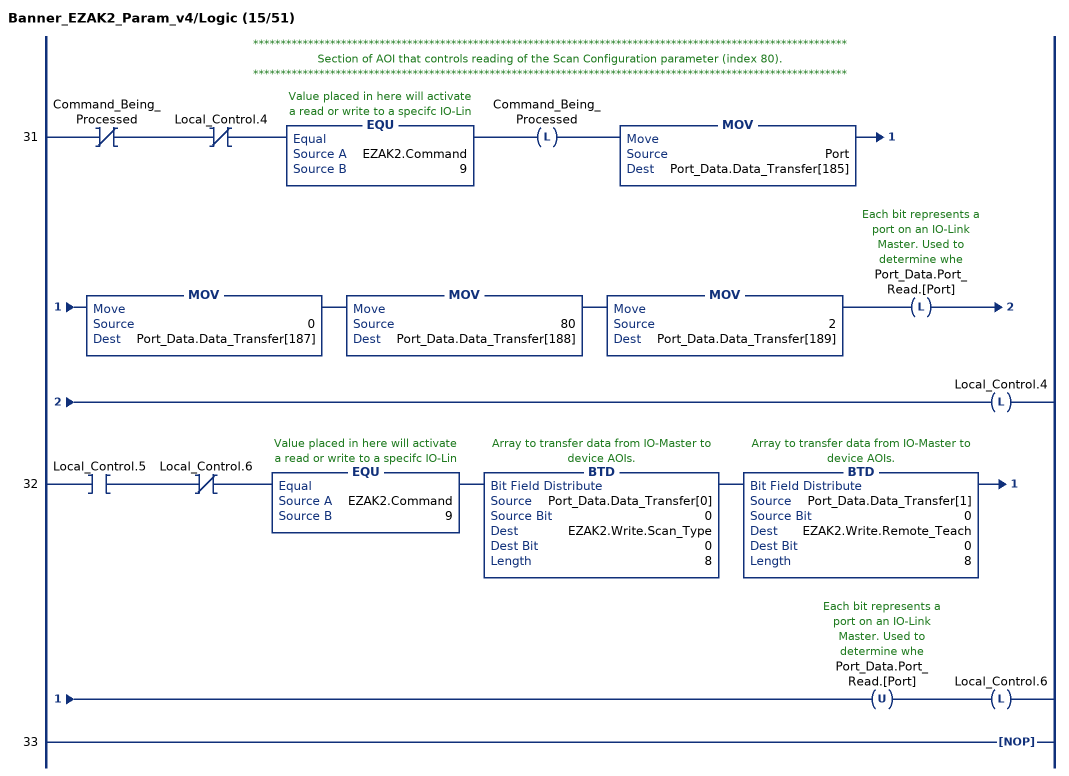
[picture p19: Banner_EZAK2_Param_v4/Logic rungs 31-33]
   // ************************************************************************************************************
   // Section of AOI that controls reading of the Scan Configuration parameter (index 80).
   // ************************************************************************************************************
   31: XIO(Command_Being_Processed)XIO(Local_Control.4)EQU(EZAK2.Command,9)OTL(Command_Being_Processed)MOV(Port,Port_Data.Data_Transfer[185])MOV(0,Port_Data.Data_Transfer[187])MOV(80,Port_Data.Data_Transfer[188])MOV(2,Port_Data.Data_Transfer[189])OTL(Port_Data.Port_Read.[Port])OTL(Local_Control.4);
   32: XIC(Local_Control.5)XIO(Local_Control.6)EQU(EZAK2.Command,9)BTD(Port_Data.Data_Transfer[0],0,EZAK2.Write.Scan_Type,0,8)BTD(Port_Data.Data_Transfer[1],0,EZAK2.Write.Remote_Teach,0,8)OTU(Port_Data.Port_Read.[Port])OTL(Local_Control.6);
   33: NOP();
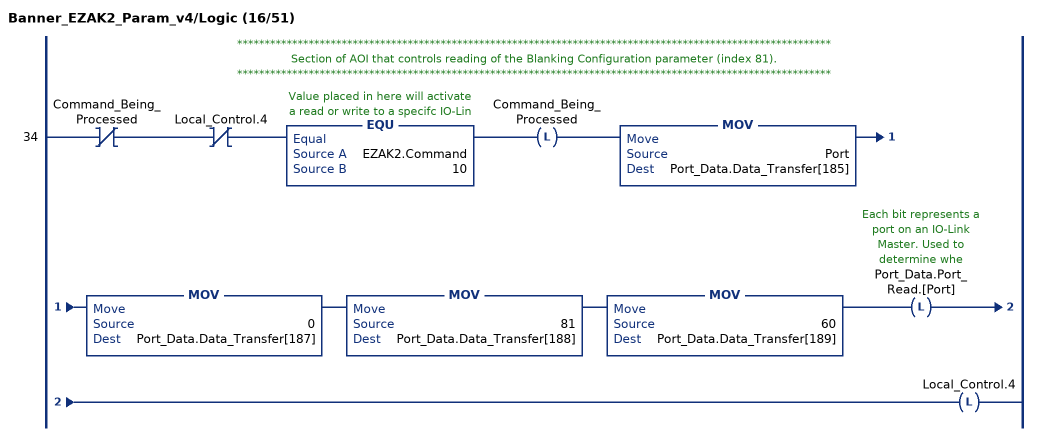
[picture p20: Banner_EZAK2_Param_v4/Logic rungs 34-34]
   // ************************************************************************************************************
   // Section of AOI that controls reading of the Blanking Configuration parameter (index 81).
   // ************************************************************************************************************
   34: XIO(Command_Being_Processed)XIO(Local_Control.4)EQU(EZAK2.Command,10)OTL(Command_Being_Processed)MOV(Port,Port_Data.Data_Transfer[185])MOV(0,Port_Data.Data_Transfer[187])MOV(81,Port_Data.Data_Transfer[188])MOV(60,Port_Data.Data_Transfer[189])OTL(Port_Data.Port_Read.[Port])OTL(Local_Control.4);
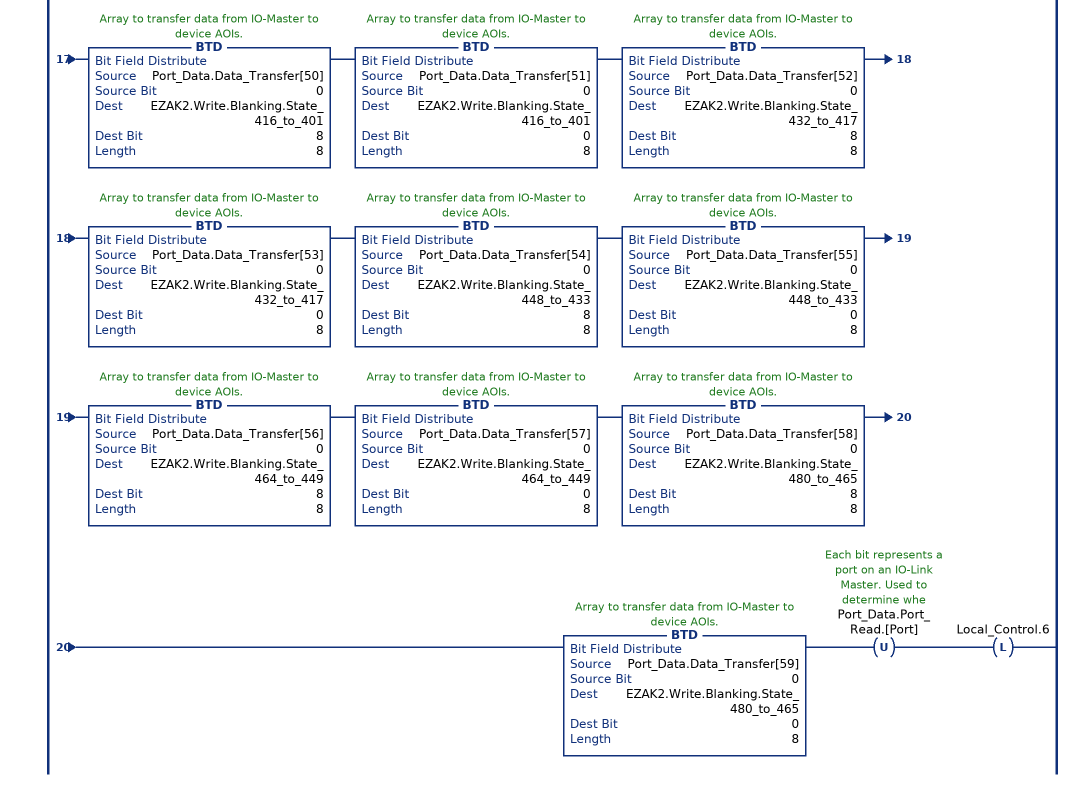
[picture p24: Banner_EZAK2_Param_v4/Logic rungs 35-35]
   35: XIC(Local_Control.5)XIO(Local_Control.6)EQU(EZAK2.Command,10)BTD(Port_Data.Data_Transfer[0],0,EZAK2.Write.Blanking.State_16_to_1,8,8)BTD(Port_Data.Data_Transfer[1],0,EZAK2.Write.Blanking.State_16_to_1,0,8)BTD(Port_Data.Data_Transfer[2],0,EZAK2.Write.Blanking.State_32_to_17,8,8)BTD(Port_Data.Data_Transfer[3],0,EZAK2.Write.Blanking.State_32_to_17,0,8)BTD(Port_Data.Data_Transfer[4],0,EZAK2.Write.Blanking.State_48_to_33,8,8)BTD(Port_Data.Data_Transfer[5],0,EZAK2.Write.Blanking.State_48_to_33,0,8)BTD(Port_Data.Data_Transfer[6],0,EZAK2.Write.Blanking.State_64_to_49,8,8)BTD(Port_Data.Data_Transfer[7],0,EZAK2.Write.Blanking.State_64_to_49,0,8)BTD(Port_Data.Data_Transfer[8],0,EZAK2.Write.Blanking.State_80_to_65,8,8)BTD(Port_Data.Data_Transfer[9],0,EZAK2.Write.Blanking.State_80_to_65,0,8)BTD(Port_Data.Data_Transfer[10],0,EZAK2.Write.Blanking.State_96_to_81,8,8)BTD(Port_Data.Data_Transfer[11],0,EZAK2.Write.Blanking.State_96_to_81,0,8)BTD(Port_Data.Data_Transfer[12],0,EZAK2.Write.Blanking.State_112_to_97,8,8)BTD(Port_Data.Data_Transfer[13],0,EZAK2.Write.Blanking.State_112_to_97,0,8)BTD(Port_Data.Data_Transfer[14],0,EZAK2.Write.Blanking.State_128_to_113,8,8)BTD(Port_Data.Data_Transfer[15],0,EZAK2.Write.Blanking.State_128_to_113,0,8)BTD(Port_Data.Data_Transfer[16],0,EZAK2.Write.Blanking.State_144_to_129,8,8)BTD(Port_Data.Data_Transfer[17],0,EZAK2.Write.Blanking.State_144_to_129,0,8)BTD(Port_Data.Data_Transfer[18],0,EZAK2.Write.Blanking.State_160_to_145,8,8)BTD(Port_Data.Data_Transfer[19],0,EZAK2.Write.Blanking.State_160_to_145,0,8)BTD(Port_Data.Data_Transfer[20],0,EZAK2.Write.Blanking.State_176_to_161,8,8)BTD(Port_Data.Data_Transfer[21],0,EZAK2.Write.Blanking.State_176_to_161,0,8)BTD(Port_Data.Data_Transfer[22],0,EZAK2.Write.Blanking.State_192_to_177,8,8)BTD(Port_Data.Data_Transfer[23],0,EZAK2.Write.Blanking.State_192_to_177,0,8)BTD(Port_Data.Data_Transfer[24],0,EZAK2.Write.Blanking.State_208_to_193,8,8)BTD(Port_Data.Data_Transfer[25],0,EZAK2.Write.Blanking.State_208_to_193,0,8)BTD(Port_Data.Data_Transfer[26],0,EZAK2.Write.Blanking.State_224_to_209,8,8)BTD(Port_Data.Data_Transfer[27],0,EZAK2.Write.Blanking.State_224_to_209,0,8)BTD(Port_Data.Data_Transfer[28],0,EZAK2.Write.Blanking.State_240_to_225,8,8)BTD(Port_Data.Data_Transfer[29],0,EZAK2.Write.Blanking.State_240_to_225,0,8)BTD(Port_Data.Data_Transfer[30],0,EZAK2.Write.Blanking.State_256_to_241,8,8)BTD(Port_Data.Data_Transfer[31],0,EZAK2.Write.Blanking.State_256_to_241,0,8)BTD(Port_Data.Data_Transfer[32],0,EZAK2.Write.Blanking.State_272_to_257,8,8)BTD(Port_Data.Data_Transfer[33],0,EZAK2.Write.Blanking.State_272_to_257,0,8)BTD(Port_Data.Data_Transfer[34],0,EZAK2.Write.Blanking.State_288_to_273,8,8)BTD(Port_Data.Data_Transfer[35],0,EZAK2.Write.Blanking.State_288_to_273,0,8)BTD(Port_Data.Data_Transfer[36],0,EZAK2.Write.Blanking.State_304_to_289,8,8)BTD(Port_Data.Data_Transfer[37],0,EZAK2.Write.Blanking.State_304_to_289,0,8)BTD(Port_Data.Data_Transfer[38],0,EZAK2.Write.Blanking.State_320_to_305,8,8)BTD(Port_Data.Data_Transfer[39],0,EZAK2.Write.Blanking.State_320_to_305,0,8)BTD(Port_Data.Data_Transfer[40],0,EZAK2.Write.Blanking.State_336_to_321,8,8)BTD(Port_Data.Data_Transfer[41],0,EZAK2.Write.Blanking.State_336_to_321,0,8)BTD(Port_Data.Data_Transfer[42],0,EZAK2.Write.Blanking.State_352_to_337,8,8)BTD(Port_Data.Data_Transfer[43],0,EZAK2.Write.Blanking.State_352_to_337,0,8)BTD(Port_Data.Data_Transfer[44],0,EZAK2.Write.Blanking.State_368_to_353,8,8)BTD(Port_Data.Data_Transfer[45],0,EZAK2.Write.Blanking.State_368_to_353,0,8)BTD(Port_Data.Data_Transfer[46],0,EZAK2.Write.Blanking.State_384_to_369,8,8)BTD(Port_Data.Data_Transfer[47],0,EZAK2.Write.Blanking.State_384_to_369,0,8)BTD(Port_Data.Data_Transfer[48],0,EZAK2.Write.Blanking.State_400_to_385,8,8)BTD(Port_Data.Data_Transfer[49],0,EZAK2.Write.Blanking.State_400_to_385,0,8)BTD(Port_Data.Data_Transfer[50],0,EZAK2.Write.Blanking.State_416_to_401,8,8)BTD(Port_Data.Data_Transfer[51],0,EZAK2.Write.Blanking.State_416_to_401,0,8)BTD(Port_Data.Data_Transfer[52],0,EZAK2.Write.Blanking.State_432_to_417,8,8)BTD(Port_Data.Data_Transfer[53],0,EZAK2.Write.Blanking.State_432_to_417,0,8)BTD(Port_Data.Data_Transfer[54],0,EZAK2.Write.Blanking.State_448_to_433,8,8)BTD(Port_Data.Data_Transfer[55],0,EZAK2.Write.Blanking.State_448_to_433,0,8)BTD(Port_Data.Data_Transfer[56],0,EZAK2.Write.Blanking.State_464_to_449,8,8)BTD(Port_Data.Data_Transfer[57],0,EZAK2.Write.Blanking.State_464_to_449,0,8)BTD(Port_Data.Data_Transfer[58],0,EZAK2.Write.Blanking.State_480_to_465,8,8)BTD(Port_Data.Data_Transfer[59],0,EZAK2.Write.Blanking.State_480_to_465,0,8)OTU(Port_Data.Port_Read.[Port])OTL(Local_Control.6);
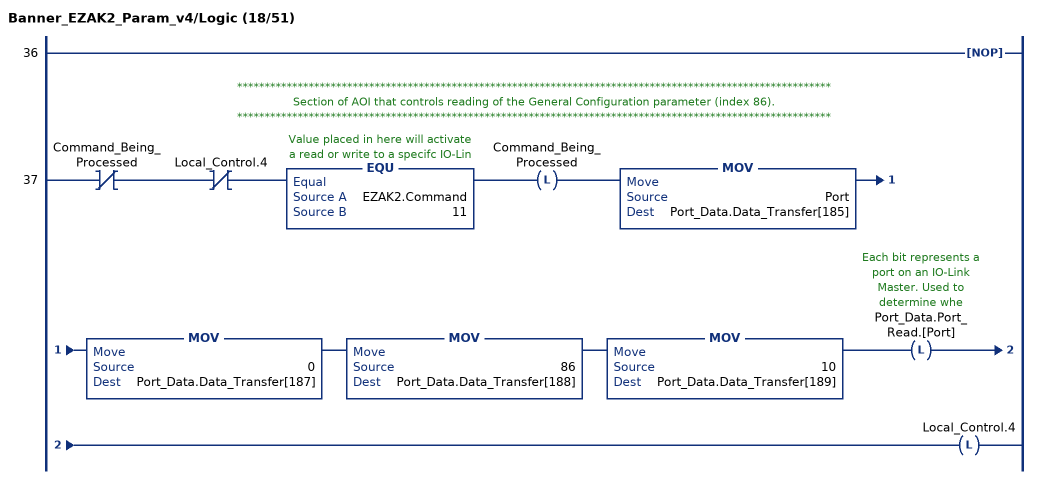
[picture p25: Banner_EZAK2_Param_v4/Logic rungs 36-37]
   36: NOP();
   // ************************************************************************************************************
   // Section of AOI that controls reading of the General Configuration parameter (index 86).
   // ************************************************************************************************************
   37: XIO(Command_Being_Processed)XIO(Local_Control.4)EQU(EZAK2.Command,11)OTL(Command_Being_Processed)MOV(Port,Port_Data.Data_Transfer[185])MOV(0,Port_Data.Data_Transfer[187])MOV(86,Port_Data.Data_Transfer[188])MOV(10,Port_Data.Data_Transfer[189])OTL(Port_Data.Port_Read.[Port])OTL(Local_Control.4);
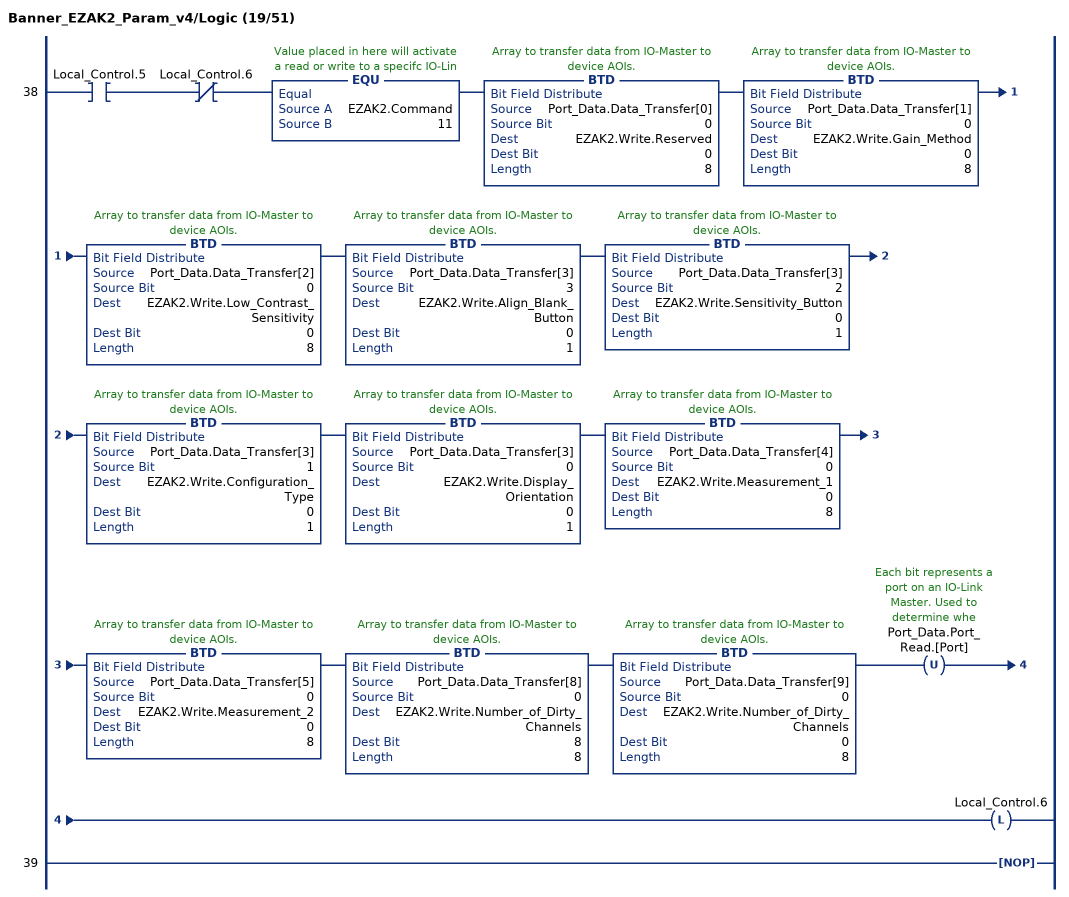
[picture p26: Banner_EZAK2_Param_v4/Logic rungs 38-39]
   38: XIC(Local_Control.5)XIO(Local_Control.6)EQU(EZAK2.Command,11)BTD(Port_Data.Data_Transfer[0],0,EZAK2.Write.Reserved,0,8)BTD(Port_Data.Data_Transfer[1],0,EZAK2.Write.Gain_Method,0,8)BTD(Port_Data.Data_Transfer[2],0,EZAK2.Write.Low_Contrast_Sensitivity,0,8)BTD(Port_Data.Data_Transfer[3],3,EZAK2.Write.Align_Blank_Button,0,1)BTD(Port_Data.Data_Transfer[3],2,EZAK2.Write.Sensitivity_Button,0,1)BTD(Port_Data.Data_Transfer[3],1,EZAK2.Write.Configuration_Type,0,1)BTD(Port_Data.Data_Transfer[3],0,EZAK2.Write.Display_Orientation,0,1)BTD(Port_Data.Data_Transfer[4],0,EZAK2.Write.Measurement_1,0,8)BTD(Port_Data.Data_Transfer[5],0,EZAK2.Write.Measurement_2,0,8)BTD(Port_Data.Data_Transfer[8],0,EZAK2.Write.Number_of_Dirty_Channels,8,8)BTD(Port_Data.Data_Transfer[9],0,EZAK2.Write.Number_of_Dirty_Channels,0,8)OTU(Port_Data.Port_Read.[Port])OTL(Local_Control.6);
   39: NOP();
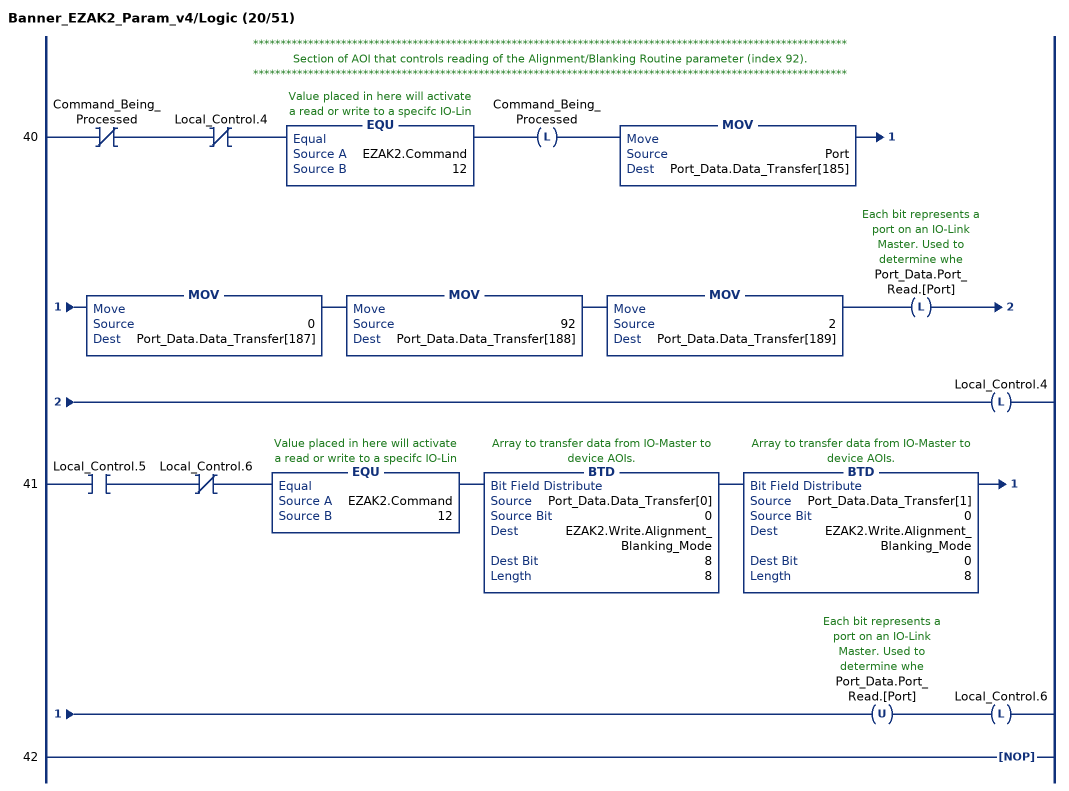
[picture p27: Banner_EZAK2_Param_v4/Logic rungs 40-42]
   // ************************************************************************************************************
   // Section of AOI that controls reading of the Alignment/Blanking Routine parameter (index 92).
   // ************************************************************************************************************
   40: XIO(Command_Being_Processed)XIO(Local_Control.4)EQU(EZAK2.Command,12)OTL(Command_Being_Processed)MOV(Port,Port_Data.Data_Transfer[185])MOV(0,Port_Data.Data_Transfer[187])MOV(92,Port_Data.Data_Transfer[188])MOV(2,Port_Data.Data_Transfer[189])OTL(Port_Data.Port_Read.[Port])OTL(Local_Control.4);
   41: XIC(Local_Control.5)XIO(Local_Control.6)EQU(EZAK2.Command,12)BTD(Port_Data.Data_Transfer[0],0,EZAK2.Write.Alignment_Blanking_Mode,8,8)BTD(Port_Data.Data_Transfer[1],0,EZAK2.Write.Alignment_Blanking_Mode,0,8)OTU(Port_Data.Port_Read.[Port])OTL(Local_Control.6);
   42: NOP();
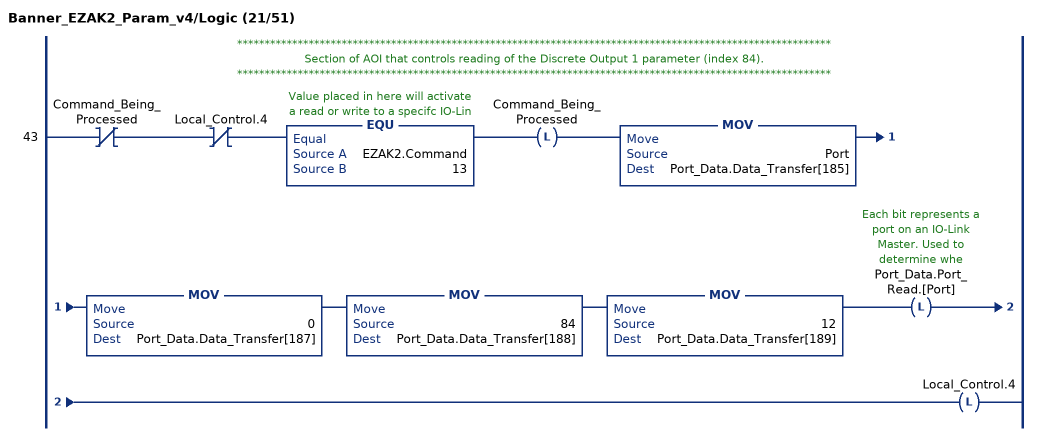
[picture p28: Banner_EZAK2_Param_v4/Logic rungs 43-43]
   // ************************************************************************************************************
   // Section of AOI that controls reading of the Discrete Output 1 parameter (index 84).
   // ************************************************************************************************************
   43: XIO(Command_Being_Processed)XIO(Local_Control.4)EQU(EZAK2.Command,13)OTL(Command_Being_Processed)MOV(Port,Port_Data.Data_Transfer[185])MOV(0,Port_Data.Data_Transfer[187])MOV(84,Port_Data.Data_Transfer[188])MOV(12,Port_Data.Data_Transfer[189])OTL(Port_Data.Port_Read.[Port])OTL(Local_Control.4);
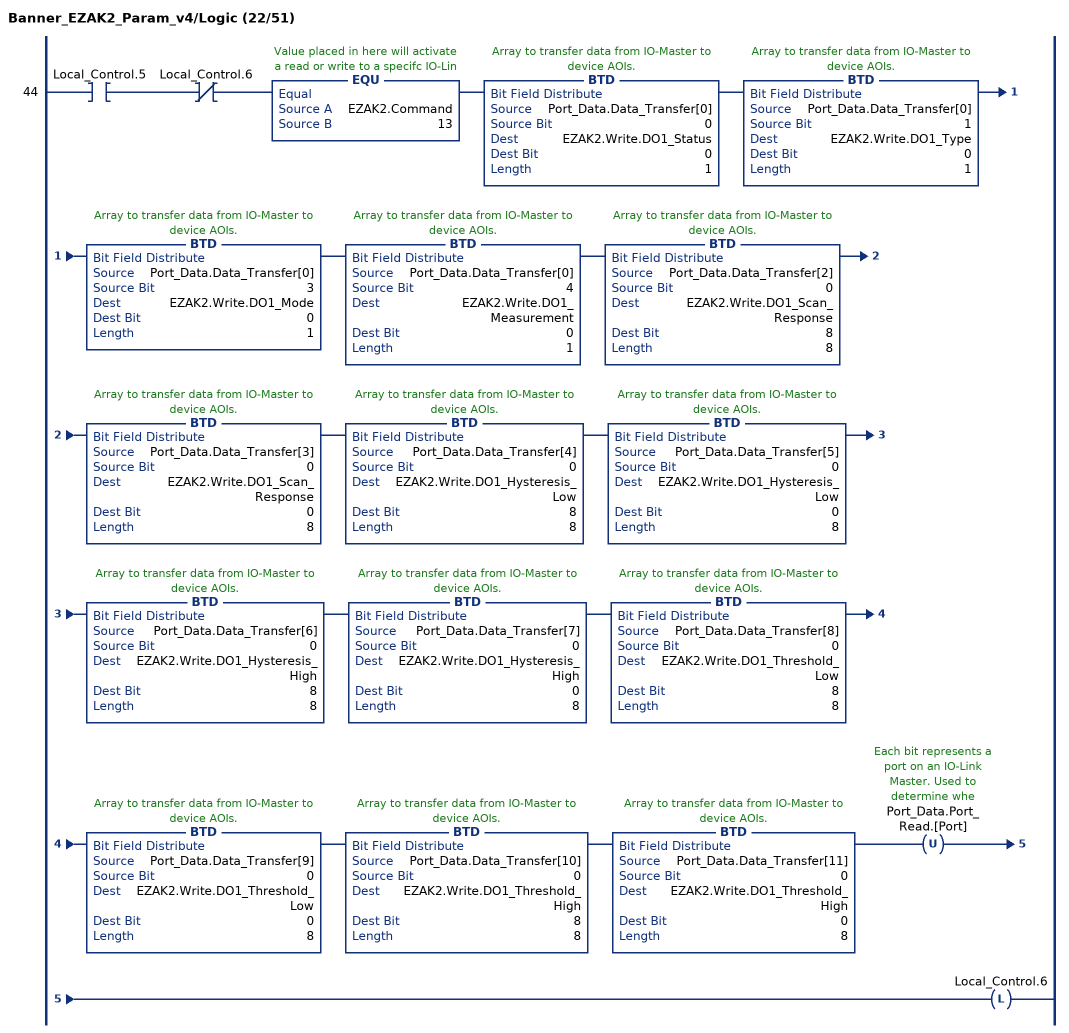
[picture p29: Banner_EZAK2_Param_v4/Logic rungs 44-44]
   44: XIC(Local_Control.5)XIO(Local_Control.6)EQU(EZAK2.Command,13)BTD(Port_Data.Data_Transfer[0],0,EZAK2.Write.DO1_Status,0,1)BTD(Port_Data.Data_Transfer[0],1,EZAK2.Write.DO1_Type,0,1)BTD(Port_Data.Data_Transfer[0],3,EZAK2.Write.DO1_Mode,0,1)BTD(Port_Data.Data_Transfer[0],4,EZAK2.Write.DO1_Measurement,0,1)BTD(Port_Data.Data_Transfer[2],0,EZAK2.Write.DO1_Scan_Response,8,8)BTD(Port_Data.Data_Transfer[3],0,EZAK2.Write.DO1_Scan_Response,0,8)BTD(Port_Data.Data_Transfer[4],0,EZAK2.Write.DO1_Hysteresis_Low,8,8)BTD(Port_Data.Data_Transfer[5],0,EZAK2.Write.DO1_Hysteresis_Low,0,8)BTD(Port_Data.Data_Transfer[6],0,EZAK2.Write.DO1_Hysteresis_High,8,8)BTD(Port_Data.Data_Transfer[7],0,EZAK2.Write.DO1_Hysteresis_High,0,8)BTD(Port_Data.Data_Transfer[8],0,EZAK2.Write.DO1_Threshold_Low,8,8)BTD(Port_Data.Data_Transfer[9],0,EZAK2.Write.DO1_Threshold_Low,0,8)BTD(Port_Data.Data_Transfer[10],0,EZAK2.Write.DO1_Threshold_High,8,8)BTD(Port_Data.Data_Transfer[11],0,EZAK2.Write.DO1_Threshold_High,0,8)OTU(Port_Data.Port_Read.[Port])OTL(Local_Control.6);
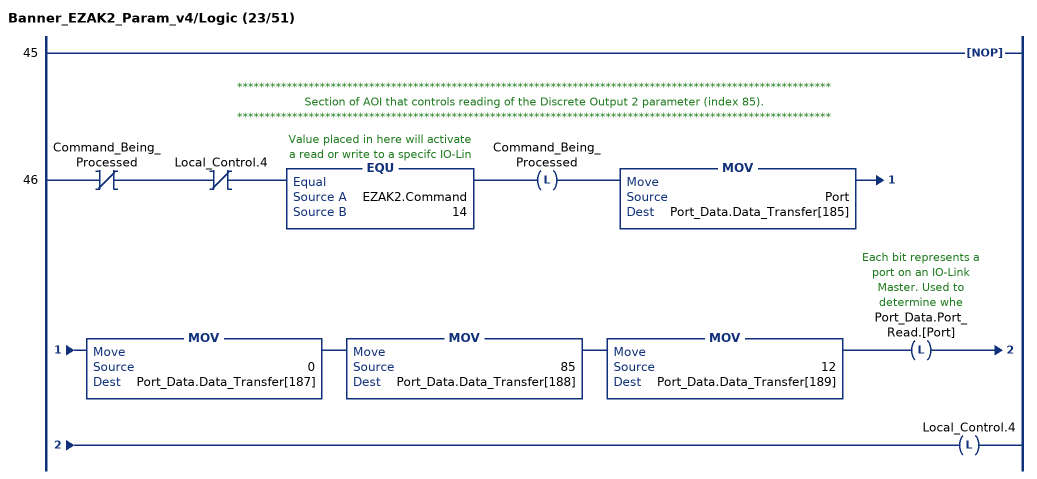
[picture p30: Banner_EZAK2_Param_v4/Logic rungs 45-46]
   45: NOP();
   // ************************************************************************************************************
   // Section of AOI that controls reading of the Discrete Output 2 parameter (index 85).
   // ************************************************************************************************************
   46: XIO(Command_Being_Processed)XIO(Local_Control.4)EQU(EZAK2.Command,14)OTL(Command_Being_Processed)MOV(Port,Port_Data.Data_Transfer[185])MOV(0,Port_Data.Data_Transfer[187])MOV(85,Port_Data.Data_Transfer[188])MOV(12,Port_Data.Data_Transfer[189])OTL(Port_Data.Port_Read.[Port])OTL(Local_Control.4);
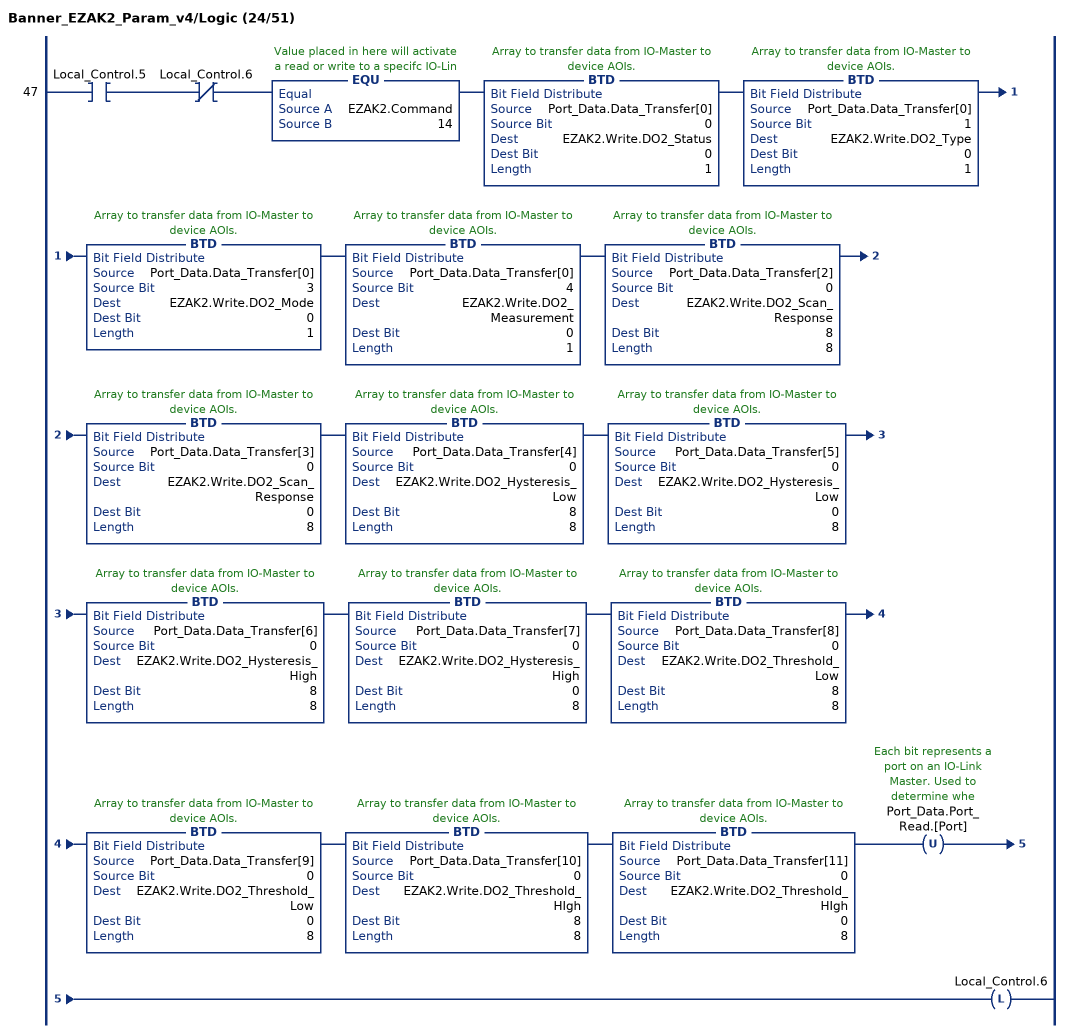
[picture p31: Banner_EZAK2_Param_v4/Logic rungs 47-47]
   47: XIC(Local_Control.5)XIO(Local_Control.6)EQU(EZAK2.Command,14)BTD(Port_Data.Data_Transfer[0],0,EZAK2.Write.DO2_Status,0,1)BTD(Port_Data.Data_Transfer[0],1,EZAK2.Write.DO2_Type,0,1)BTD(Port_Data.Data_Transfer[0],3,EZAK2.Write.DO2_Mode,0,1)BTD(Port_Data.Data_Transfer[0],4,EZAK2.Write.DO2_Measurement,0,1)BTD(Port_Data.Data_Transfer[2],0,EZAK2.Write.DO2_Scan_Response,8,8)BTD(Port_Data.Data_Transfer[3],0,EZAK2.Write.DO2_Scan_Response,0,8)BTD(Port_Data.Data_Transfer[4],0,EZAK2.Write.DO2_Hysteresis_Low,8,8)BTD(Port_Data.Data_Transfer[5],0,EZAK2.Write.DO2_Hysteresis_Low,0,8)BTD(Port_Data.Data_Transfer[6],0,EZAK2.Write.DO2_Hysteresis_High,8,8)BTD(Port_Data.Data_Transfer[7],0,EZAK2.Write.DO2_Hysteresis_High,0,8)BTD(Port_Data.Data_Transfer[8],0,EZAK2.Write.DO2_Threshold_Low,8,8)BTD(Port_Data.Data_Transfer[9],0,EZAK2.Write.DO2_Threshold_Low,0,8)BTD(Port_Data.Data_Transfer[10],0,EZAK2.Write.DO2_Threshold_HIgh,8,8)BTD(Port_Data.Data_Transfer[11],0,EZAK2.Write.DO2_Threshold_HIgh,0,8)OTU(Port_Data.Port_Read.[Port])OTL(Local_Control.6);
